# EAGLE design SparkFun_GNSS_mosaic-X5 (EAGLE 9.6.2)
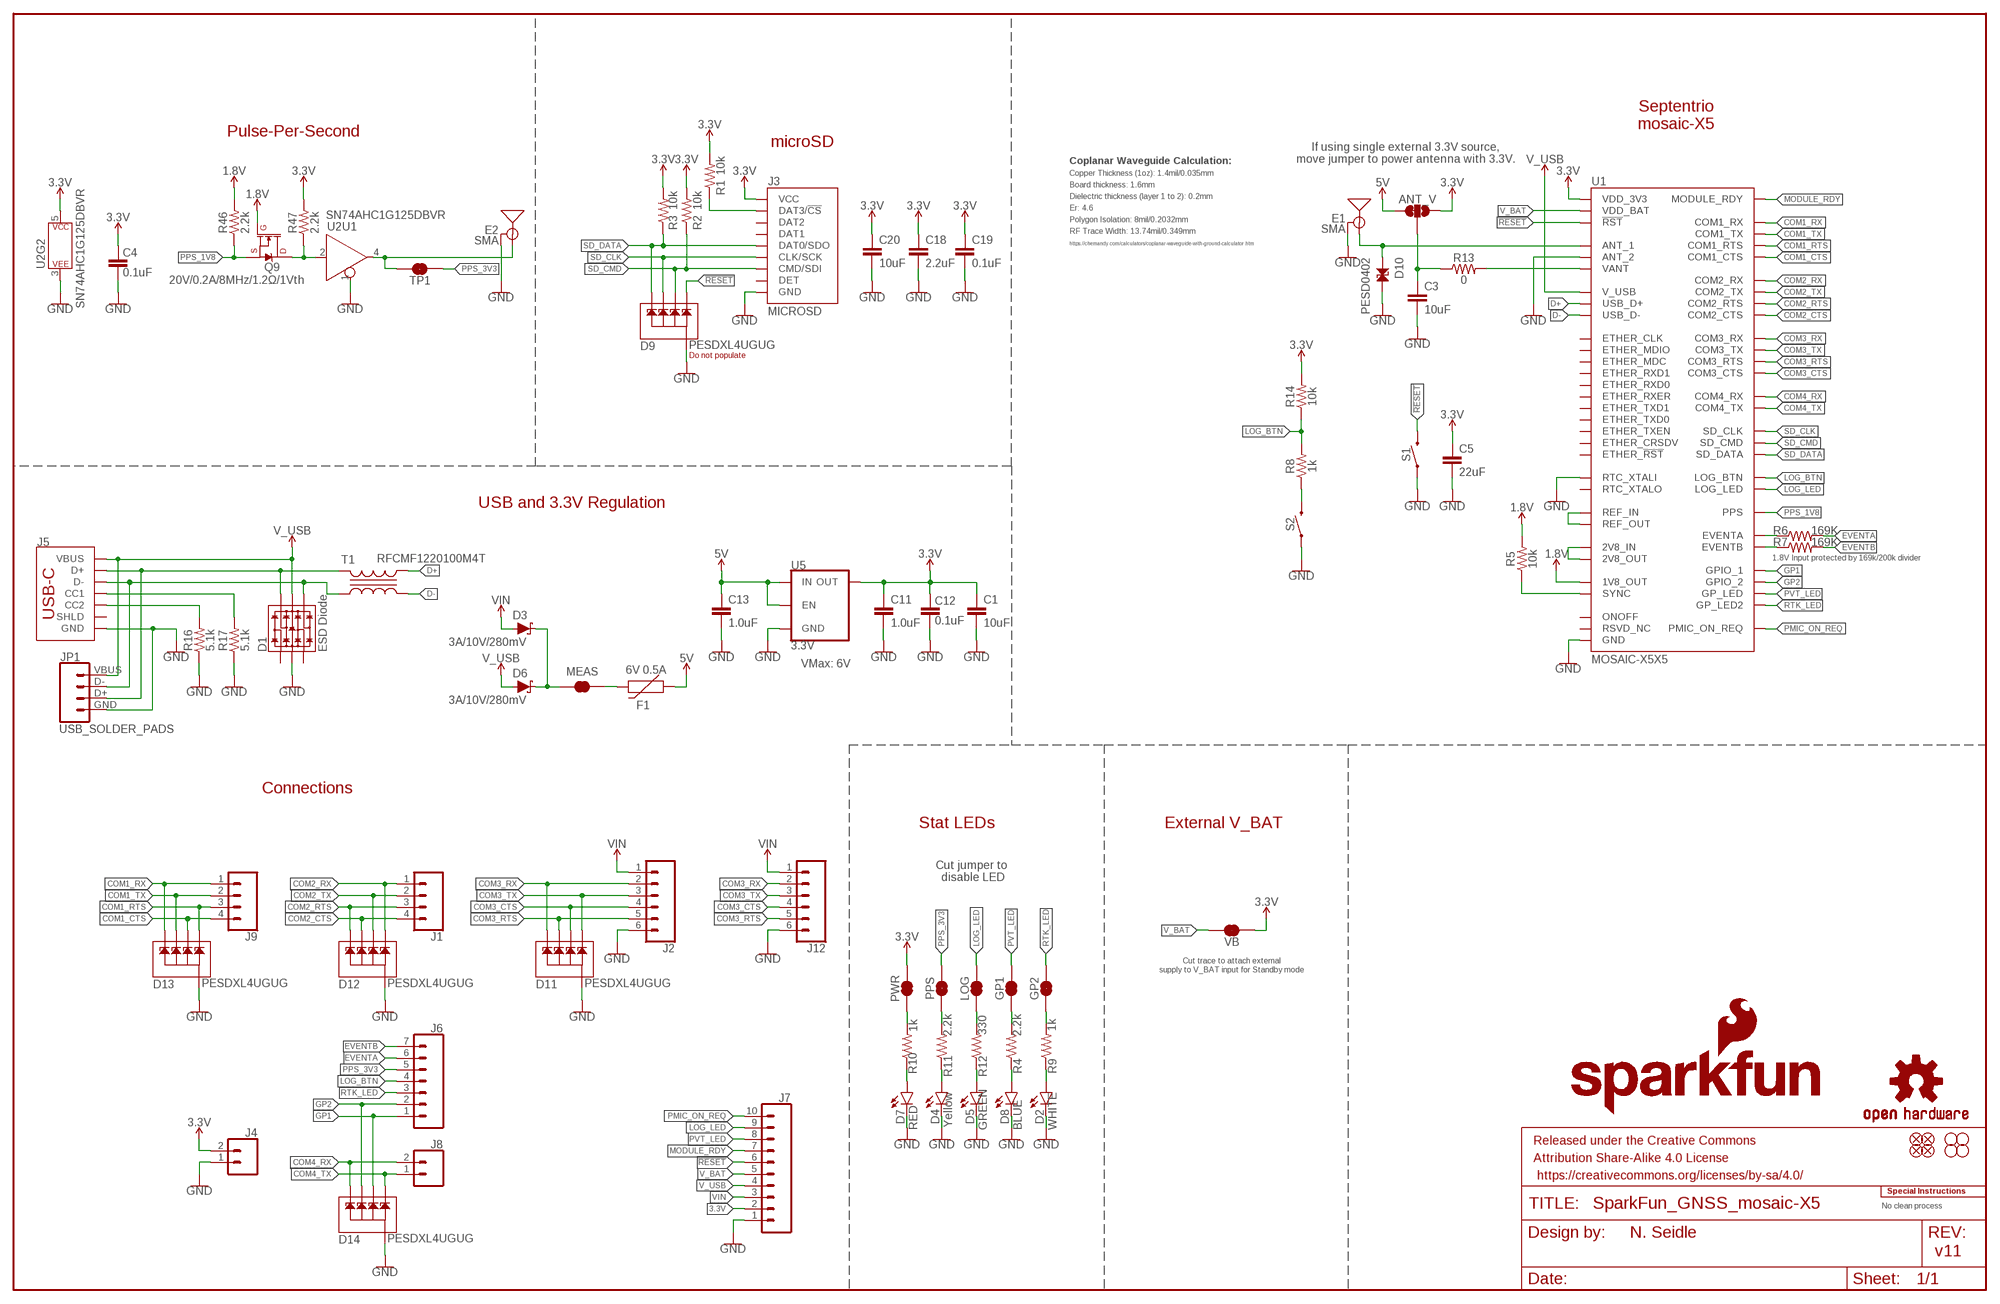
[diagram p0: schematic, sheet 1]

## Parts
ANT_V  JUMPER-SMT_3_1-NC_TRACE_SILK  [SMT-JUMPER_3_1-NC_TRACE_SILK]
C1  10uF  10UF-0603-6.3V-20%  [0603]
C3  10uF  10UF-0603-6.3V-20%  [0603]
C4  0.1uF  0.1UF-0603-25V-5%  [0603]
C5  22uF  22UF-0603-6.3V-20%  [0603]
C11  1.0uF  1.0UF-0603-16V-10%  [0603]
C12  0.1uF  0.1UF-0603-25V-5%  [0603]
C13  1.0uF  1.0UF-0603-16V-10%  [0603]
C18  2.2uF  2.2UF-0603-10V-20%  [0603]
C19  0.1uF  0.1UF-0603-25V-5%  [0603]
C20  10uF  10UF-0603-6.3V-20%  [0603]
D1  ESD Diode  TVS_DIODE_ARRAY_DT1042-04SO-7  [SOT-23-6]
D2  WHITE  LED-WHITE0603  [LED-0603]
D3  3A/10V/280mV  DIODE-SCHOTTKY-BAT60A  [SOD-323]
D4  Yellow  LED-YELLOW0603  [LED-0603]
D5  GREEN  LED-GREEN0603  [LED-0603]
D6  3A/10V/280mV  DIODE-SCHOTTKY-BAT60A  [SOD-323]
D7  RED  LED-RED0603  [LED-0603]
D8  BLUE  LED-BLUE0603  [LED-0603]
D9  PESDXL4UGUG  [SOT353]
D10  PESD0402  PESD0402-0402T  [0402-TIGHT]
D11  PESDXL4UGUG  [SOT353]
D12  PESDXL4UGUG  [SOT353]
D13  PESDXL4UGUG  [SOT353]
D14  PESDXL4UGUG  [SOT353]
E1  SMA  ANTENNA-SMA-GROUNDEDEDGE_SMA  [SMA-EDGE]
E2  SMA  ANTENNA-SMA-GROUNDEDEDGE_SMA  [SMA-EDGE]
F1  6V 0.5A  PPTC_6V500MA  [0805]
FRAME2  FRAME-LEDGER  [CREATIVE_COMMONS]
GP1  JUMPER-SMT_2_NC_TRACE_SILK  [SMT-JUMPER_2_NC_TRACE_SILK]
GP2  JUMPER-SMT_2_NC_TRACE_SILK  [SMT-JUMPER_2_NC_TRACE_SILK]
H1  STAND-OFF  [STAND-OFF]
H2  STAND-OFF  [STAND-OFF]
H3  STAND-OFF  [STAND-OFF]
H4  STAND-OFF  [STAND-OFF]
J1  CONN_041X04_NO_SILK_NO_POP  [1X04_NO_SILK]
J2  CONN_06JST-SMD-LOCKING  [JST-6-SMD-1.25MM-LOCKING]
J3  MICROSD  MICRO-SD-PUSH-PUSH-EXT-PIN  [MICROSD-EXTERNALPIN]
J4  CONN_021X02_NO_SILK  [1X02_NO_SILK]
J5  USB Female Type C Connector  USB_C_4-LAYER_PADS  [USB-C-16P_4LAYER-PADS]
J6  CONN_07NO_SILK  [1X07_NO_SILK]
J7  CONN_10NO_SILK_PTH_FEMALE  [1X10_NO_SILK]
J8  CONN_021X02_NO_SILK  [1X02_NO_SILK]
J9  CONN_041X04_NO_SILK_NO_POP  [1X04_NO_SILK]
J12  CONN_06PAD  [1X06_SOLDER_PADS]
JP1  USB_SOLDER_PADS  [USB-SOLDER-PADS]
JP21  FIDUCIALUFIDUCIAL  [FIDUCIAL-MICRO]
JP61  FIDUCIALUFIDUCIAL  [FIDUCIAL-MICRO]
JP71  FIDUCIALUFIDUCIAL  [FIDUCIAL-MICRO]
JP81  FIDUCIALUFIDUCIAL  [FIDUCIAL-MICRO]
LOG  JUMPER-SMT_2_NC_TRACE_SILK  [SMT-JUMPER_2_NC_TRACE_SILK]
LOGO2  OSHW-LOGOMINI  [OSHW-LOGO-MINI]
LOGO4  SFE_LOGO_NAME_FLAME10_MM  [SFE_LOGO_NAME_FLAME_10MM]
MEAS  JUMPER-COMBO_2_NC_TRACE  [COMBO-JUMPER_2_NC_TRACE]
PPS  JUMPER-SMT_2_NC_TRACE_SILK  [SMT-JUMPER_2_NC_TRACE_SILK]
PWR  JUMPER-SMT_2_NC_TRACE_SILK  [SMT-JUMPER_2_NC_TRACE_SILK]
Q9  20V/0.2A/8MHz/1.2Ω/1Vth  MOSFET-NCH-RE1C002UNTCL  [SOT-416FL]
R1  10k  10KOHM-0603-1/10W-1%  [0603]
R2  10k  10KOHM-0603-1/10W-1%  [0603]
R3  10k  10KOHM-0603-1/10W-1%  [0603]
R4  2.2k  2.2KOHM-0603-1/10W-1%  [0603]
R5  10k  10KOHM-0603-1/10W-1%  [0603]
R6  169K  169KOHM  [0603]
R7  169K  169KOHM  [0603]
R8  1k  1KOHM-0603-1/10W-1%  [0603]
R9  1k  1KOHM-0603-1/10W-1%  [0603]
R10  1k  1KOHM-0603-1/10W-1%  [0603]
R11  2.2k  2.2KOHM-0603-1/10W-1%  [0603]
R12  330  330OHM-0603-1/10W-1%  [0603]
R13  0  0OHM-0603-1/10W  [0603]
R14  10k  10KOHM-0603-1/10W-1%  [0603]
R16  5.1k  5.1KOHM5.1KOHM-0603-1/10W-1%  [0603]
R17  5.1k  5.1KOHM5.1KOHM-0603-1/10W-1%  [0603]
R46  2.2k  2.2KOHM-0603-1/10W-1%  [0603]
R47  2.2k  2.2KOHM-0603-1/10W-1%  [0603]
S1  MOMENTARY-SWITCH-SPST-SMD-4.6X2.8MM  [TACTILE_SWITCH_SMD_4.6X2.8MM]
S2  MOMENTARY-SWITCH-SPST-SMD-5.2-TALL-REDUNDANT  [TACTILE_SWITCH_SMD_5.2MM]
T1  RFCMF1220100M4T  TRANSFORMER0508  [RFCMF1220100M4T]
TP1  JUMPER-SMT_2_NC_TRACE_SILK  [SMT-JUMPER_2_NC_TRACE_SILK]
U1  MOSAIC-X5X5  [MOSAIC_LGA]
U2  SN74AHC1G125DBVR  74AHC1G125SN74AHC1G125DBVR  [SOT23-5]
U5  3.3V  V_REG_AP2112K-3.3V  [SOT23-5]
U$2  SPECIAL_INSTRUCTIONS-ORDERING  [ORDERING_INSTRUCTIONS]
VB  JUMPER-SMT_2_NC_TRACE_SILK  [SMT-JUMPER_2_NC_TRACE_SILK]

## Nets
1.8V: Q9.1(G) R5.2 R46.2 U1.AC4(1V8_OUT)
3.3V [power]: ANT_V.1 C1.1 C4.2 C5.1 C11.1 C12.2 C18.1 C19.1 C20.1 J3.4(VCC) J4.2 J7.2 PWR.2 R1.2 R2.2 R3.2 R14.2 R47.2 U1.A18(VDD_3V3) U1.A19(VDD_3V3) U1.A20(VDD_3V3) U1.B18(VDD_3V3) U1.B19(VDD_3V3) U1.B20(VDD_3V3) U1.C18(VDD_3V3) U1.C19(VDD_3V3) U1.C20(VDD_3V3) U2.5(P$V+) U5.5(OUT) VB.1
5V: ANT_V.3 C13.1 F1.1 U5.1(IN) U5.3(EN)
!RESET!: D9.3 J7.6 S1.3 S1.4 U1.A11(!RST!)
ANT_V: ANT_V.2 C3.1 R13.1
CC1: J5.A5(CC1) R17.2
CC2: J5.B5(CC2) R16.2
COM1_CTS: D13.4 J9.4 U1.E1(COM1_CTS)
COM1_RTS: D13.3 J9.3 U1.C1(COM1_RTS)
COM1_RX: D13.1 J9.1 U1.B1(COM1_RX)
COM1_TX: D13.5 J9.2 U1.D1(COM1_TX)
COM2_CTS: D12.5 J1.4 U1.J1(COM2_CTS)
COM2_RTS: D12.1 J1.3 U1.G1(COM2_RTS)
COM2_RX: D12.3 J1.1 U1.F1(COM2_RX)
COM2_TX: D12.4 J1.2 U1.H1(COM2_TX)
COM3_CTS: D11.4 J2.4 J12.4 U1.N1(COM3_CTS)
COM3_RTS: D11.5 J2.5 J12.5 U1.L1(COM3_RTS)
COM3_RX: D11.1 J2.2 J12.2 U1.K1(COM3_RX)
COM3_TX: D11.3 J2.3 J12.3 U1.M1(COM3_TX)
COM4_RX: D14.1 J8.2 U1.D3(COM4_RX)
COM4_TX: D14.3 J8.1 U1.E3(COM4_TX)
D+: T1.B2 U1.A5(USB_D+)
D-: T1.A2 U1.A6(USB_D-)
EVENTA: J6.6 R6.2
EVENTB: J6.7 R7.2
GND: C1.2 C3.2 C4.1 C5.2 C11.2 C12.1 C13.2 C18.2 C19.2 C20.2 D1.2(VSS) D2.C D4.C D5.C D7.C D8.C D9.2 D10.2 D11.2 D12.2 D13.2 D14.2 E1.GND@0(GND) E1.GND@1(GND) E1.GND@2(GND) E1.GND@3(GND) E2.GND@0(GND) E2.GND@1(GND) E2.GND@2(GND) E2.GND@3(GND) J2.6 J3.6(GND) J3.10(GND) J3.11(GND) J3.12(GND) J3.13(GND) J4.1 J5.GND J5.GND2(GND) J7.1 J12.6 JP1.GND R16.1 R17.1 S1.1 S1.2 S2.1 S2.2 U1.A3(RTC_XTALI) U1.A4(GND) U1.A7(GND) U1.A15(GND) U1.A16(GND) U1.A17(GND) U1.A21(GND) U1.A22(GND) U1.A23(GND) U1.AA13(GND) U1.AA14(GND) U1.AA15(GND) U1.AA16(GND) U1.AA17(GND) U1.AA18(GND) U1.AA19(GND) U1.AA20(GND) U1.AA21(GND) U1.AA22(GND) U1.AA23(GND) U1.AB2(GND) U1.AB3(GND) U1.AB4(GND) U1.AB5(GND) U1.AB6(GND) U1.AB7(GND) U1.AB8(GND) U1.AB13(GND) U1.AB14(GND) U1.AB15(GND) U1.AB16(GND) U1.AB17(GND) U1.AB18(GND) U1.AB19(GND) U1.AB20(GND) U1.AB21(GND) U1.AB22(GND) U1.AB23(GND) U1.AC13(GND) U1.AC15(GND) U1.AC18(GND) U1.AC19(GND) U1.AC21(GND) U1.AC22(GND) U1.AC23(GND) U1.B4(GND) U1.B5(GND) U1.B6(GND) U1.B7(GND) U1.B13(GND) U1.B17(GND) U1.B21(GND) U1.C4(GND) U1.C7(GND) U1.C15(GND) U1.C16(GND) U1.C17(GND) U1.C23(GND) U1.D2(GND) U1.D21(GND) U1.D22(GND) U1.D23(GND) U1.E2(GND) U1.E21(GND) U1.E22(GND) U1.E23(GND) U1.F21(GND) U1.F22(GND) U1.F23(GND) U1.G2(GND) U1.G21(GND) U1.G23(GND) U1.H21(GND) U1.H22(GND) U1.H23(GND) U1.J21(GND) U1.J22(GND) U1.J23(GND) U1.K2(GND) U1.K21(GND) U1.K22(GND) U1.K23(GND) U1.L21(GND) U1.L22(GND) U1.L23(GND) U1.M21(GND) U1.M22(GND) U1.N21(GND) U1.N22(GND) U1.P1(GND) U1.P2(GND) U1.P3(GND) U1.P21(GND) U1.P22(GND) U1.R3(GND) U1.R21(GND) U1.R22(GND) U1.T21(GND) U1.T22(GND) U1.T23(GND) U1.U2(GND) U1.U21(GND) U1.U22(GND) U1.U23(GND) U1.V21(GND) U1.V22(GND) U1.V23(ANT_2) U1.W21(GND) U1.W22(GND) U1.W23(GND) U1.Y2(GND) U1.Y21(GND) U1.Y22(GND) U1.Y23(GND) U2.1(U1:!EN) U2.3(P$V-) U5.2(GND)
GP1: D14.4 J6.1 U1.AA4(GPIO_1)
GP2: D14.5 J6.2 U1.L3(GPIO_2)
GPS_ANT1 [RF]: D10.1 E1.SIG(SIGNAL) U1.AC20(ANT_1)
LOG_BTN: J6.4 R8.2 R14.1 U1.K3(LOG_BTN)
LOG_LED: J7.9 LOG.2 U1.B2(LOG_LED)
MEAS: D3.C D6.C MEAS.2 MEAS.4
MODULE_RDY: J7.7 U1.A12(MODULE_RDY)
N$1: R8.1 S2.3 S2.4
N$2: D4.A R11.1
N$3: PPS.1 R11.2
N$4: F1.2 MEAS.1 MEAS.3
N$5: J3.2(DAT3/!CS!) R1.1
N$6: R6.1 U1.AC6(EVENTA)
N$7: R7.1 U1.AC7(EVENTB)
N$8: D2.A R9.1
N$9: GP2.1 R9.2
N$10: U1.AC16(REF_OUT) U1.AC17(REF_IN)
N$11: D8.A R4.1
N$12: GP1.1 R4.2
N$14: D7.A R10.1
N$15: U1.M23(2V8_IN) U1.N23(2V8_OUT)
N$16: D5.A R12.1
N$17: LOG.1 R12.2
N$20: PWR.1 R10.2
N$26: R5.1 U1.AC3(SYNC)
PMIC_ON_REQ: J7.10 U1.B16(PMIC_ON_REQ)
PPS: E2.SIG(SIGNAL) TP1.2 U2.4(U1:Y)
PPS_1V8: Q9.2(S) R46.1 U1.AC8(PPS)
PPS_3: Q9.3(D) R47.1 U2.2(U1:A)
PPS_3V3: J6.5 PPS.2 TP1.1
PVT_LED: GP1.2 J7.8 U1.A14(GP_LED)
RTK_LED: GP2.2 J6.3 U1.M3(GP_LED2)
SD_CLK: D9.5 J3.5(CLK/SCK) U1.AA1(SD_CLK)
SD_CMD: D9.4 J3.3(CMD/SDI) R2.1 U1.AB1(SD_CMD)
SD_DATA: D9.1 J3.7(DAT0/SDO) R3.1 U1.Y1(SD_DATA)
USB_D+: D1.6(IO4) J5.A6(D+) J5.B6(D+) JP1.D+ T1.B1
USB_D-: D1.4(IO3) J5.A7(D-) J5.B7(D-) JP1.D- T1.A1
V_BAT: J7.5 U1.B8(VDD_BAT) VB.2
V_USB: D1.5(VCC) D6.A J5.VBUS1(VBUS) J5.VBUS2(VBUS) J7.4 JP1.VBUS U1.A8(V_USB)
VANT: R13.2 U1.P23(VANT) U1.R23(VANT)
VIN: D3.A J2.1 J7.3 J12.1
Unconnected: D1.1(IO1) D1.3(IO2) J3.1(DAT2) J3.8(DAT1) J3.9(DET) J5.SHLD1(SHLD) J5.SHLD2(SHLD) J5.SHLD3(SHLD) J5.SHLD4(SHLD) U1.A2(RTC_XTALO) U1.A9(RSVD_NC) U1.A10(ONOFF) U1.A13(RSVD_NC) U1.AA2(ETHER_CLK) U1.AA3(RSVD_NC) U1.AA5(RSVD_NC) U1.AA6(RSVD_NC) U1.AA7(RSVD_NC) U1.AA8(RSVD_NC) U1.AA9(RSVD_NC) U1.AA10(RSVD_NC) U1.AA11(RSVD_NC) U1.AA12(RSVD_NC) U1.AB9(RSVD_NC) U1.AB10(RSVD_NC) U1.AB11(RSVD_NC) U1.AB12(RSVD_NC) U1.AC1(RSVD_NC) U1.AC2(RSVD_NC) U1.AC5(RSVD_NC) U1.AC9(RSVD_NC) U1.AC10(RSVD_NC) U1.AC11(RSVD_NC) U1.AC12(RSVD_NC) U1.AC14(RSVD_NC) U1.B3(RSVD_NC) U1.B9(RSVD_NC) U1.B10(RSVD_NC) U1.B11(RSVD_NC) U1.B12(RSVD_NC) U1.B14(RSVD_NC) U1.B15(RSVD_NC) U1.B22(RSVD_NC) U1.B23(RSVD_NC) U1.C2(RSVD_NC) U1.C3(RSVD_NC) U1.C5(RSVD_NC) U1.C6(RSVD_NC) U1.C8(RSVD_NC) U1.C9(RSVD_NC) U1.C10(RSVD_NC) U1.C11(RSVD_NC) U1.C12(RSVD_NC) U1.C13(RSVD_NC) U1.C14(RSVD_NC) U1.C21(RSVD_NC) U1.C22(RSVD_NC) U1.F2(ETHER_!RST!) U1.F3(RSVD_NC) U1.G3(RSVD_NC) U1.G22(RSVD_NC) U1.H2(ETHER_TXD1) U1.H3(RSVD_NC) U1.J2(ETHER_TXD0) U1.J3(RSVD_NC) U1.L2(ETHER_TXEN) U1.M2(ETHER_RXER) U1.N2(ETHER_CRSDV) U1.N3(RSVD_NC) U1.R1(RSVD_NC) U1.R2(ETHER_RXD0) U1.T1(RSVD_NC) U1.T2(ETHER_RXD1) U1.T3(RSVD_NC) U1.U1(RSVD_NC) U1.U3(RSVD_NC) U1.V1(RSVD_NC) U1.V2(ETHER_MDC) U1.V3(RSVD_NC) U1.W1(RSVD_NC) U1.W2(ETHER_MDIO) U1.W3(RSVD_NC) U1.Y3(RSVD_NC)

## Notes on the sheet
- Septentrio
  mosaic-X5
- Pulse-Per-Second
- microSD
- If using single external 3.3V source,
  move jumper to power antenna with 3.3V.
- Coplanar Waveguide Calculation:
- Copper Thickness (1oz): 1.4mil/0.035mm
- Board thickness: 1.6mm
- Dielectric thickness (layer 1 to 2): 0.2mm
- Er: 4.6
- Polygon Isolation: 8mil/0.2032mm
- RF Trace Width: 13.74mil/0.349mm
- https://chemandy.com/calculators/coplanar-waveguide-with-ground-calculator.htm
- Do not populate
- USB and 3.3V Regulation
- 1.8V Input protected by 169k/200k divider
- VMax: 6V
- Connections
- Stat LEDs | External V_BAT
- Cut jumper to 
  disable LED
- Cut trace to attach external
  supply to V_BAT input for Standby mode
- No clean process
- N. Seidle
- v11

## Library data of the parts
ANT_V = SparkFun-Jumpers:JUMPER-SMT_3_1-NC_TRACE: Normally closed trace jumper (1 of 2 connections) This jumper has a trace between two pads so it's normally closed (NC). The other connection is normally open (NO). Use a razor knife to open the connection. For best results follow the IPC guidelines for cutting traces: Cutout at least 0.063 mm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
C1 C3 C20 = SparkFun-Capacitors:10UF: 10.0µF ceramic capacitors; PROD_ID: CAP-11015
C4 C12 C19 = SparkFun-Capacitors:0.1UF: 0.1µF ceramic capacitors; PROD_ID: CAP-08604
C5 = SparkFun-Capacitors:22UF: 22µF ceramic capacitors; PROD_ID: CAP-14464
C11 C13 = SparkFun-Capacitors:1.0UF: 1µF ceramic capacitors; PROD_ID: CAP-00868
C18 = SparkFun-Capacitors:2.2UF: 2.2µF ceramic capacitors; PROD_ID: CAP-07888
D1 = SparkFun-DiscreteSemi:TVS_DIODE_ARRAY; PROD_ID: IC-13538
D2 = SparkFun-LED:LED-WHITE: White SMD LED; PROD_ID: DIO-09004
D3 D6 = SparkFun-DiscreteSemi:DIODE-SCHOTTKY: Schottky diode; PROD_ID: DIO-14072
D4 = SparkFun-LED:LED-YELLOW: Yellow SMD LED; PROD_ID: DIO-09003
D5 = SparkFun-LED:LED-GREEN: Green SMD LED; PROD_ID: DIO-00821
D7 = SparkFun-LED:LED-RED: Red SMD LED; PROD_ID: DIO-00819
D8 = SparkFun-LED:LED-BLUE: Blue SMD LED; PROD_ID: DIO-08575
D9 D11-D14 = SparkFun-DiscreteSemi:PESDXL4UG; PROD_ID: DIO-19494
D10 = SparkFun-DiscreteSemi:PESD0402: ESD protection diode; PROD_ID: DIO-15359
E1 E2 = SparkFun-RF:ANTENNA-SMA-GROUNDED: SMA Antenna Connector w/ Ground; PROD_ID: CONN-08289
F1 = SparkFun-Fuses:PPTC: Resettable Fuse PPTC; PROD_ID: RES-13945
FRAME2 = SparkFun-Aesthetics:FRAME-LEDGER: Schematic Frame - Ledger
GP1 GP2 LOG PPS PWR TP1 VB = SparkFun-Jumpers:JUMPER-SMT_2_NC_TRACE: Normally closed trace jumper
H1-H4 = SparkFun-Hardware:STAND-OFF: Stand Off
J1 J9 = SparkFun-Connectors:CONN_04: Multi connection point. Often used as Generic Header-pin footprint for 0.1 inch spaced/style header connections On any of the 0.1 inch spaced packages, you can populate with these: Break Away Headers - Straight (PRT-00116) Break Away Male Headers - Right Angle (PRT-00553) Female Headers (PRT-00115)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
J2 = SparkFun-Connectors:CONN_06: Multi connection point. Often used as Generic Header-pin footprint for 0.1 inch spaced/style header connections On any of the 0.1 inch spaced packages, you can populate with these: Break Away Headers - Straight (PRT-00116) Break Away Male Headers - Right Angle (PRT-00553) Female Headers (PRT-00115)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; PROD_ID: CONN-16497
J3 = SparkFun-Connectors:MICRO-SD: microSD Socket for Transflash Various sockets for µSD. tDoc lines correctly indicate media card edge positions when inserting (unlocked, locked, depressed). NOTE: CD1 and CD2 are connected internally, and the default detect state of the socket is detect pin to ground. SparkFun Products: WAV Trigger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; PROD_ID: CONN-16110
J4 J8 = SparkFun-Connectors:CONN_02: Multi connection point. Often used as Generic Header-pin footprint for 0.1 inch spaced/style header connections
J5 = SparkFun-Connectors:USB_C: USB Type C 16Pin Connector Super Speed pins not available on the 16-pin purely SMD connector so this part is best for USB 2.0 implementations. D1 and D2 are tied together enabling D+/- no matter which way the cable is plugged into the connector. The two channel configuration pins (CC1/2) are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; PROD_ID: CONN-14122
J6 = SparkFun-Connectors:CONN_07: Multi connection point. Often used as Generic Header-pin footprint for 0.1 inch spaced/style header connections On any of the 0.1 inch spaced packages, you can populate with these: Break Away Headers - Straight (PRT-00116) Break Away Male Headers - Right Angle (PRT-00553) Female Headers (PRT-00115)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
J7 = SparkFun-Connectors:CONN_10: Multi connection point. Often used as Generic Header-pin footprint for 0.1 inch spaced/style header connections On any of the 0.1 inch spaced packages, you can populate with these: Break Away Headers - Straight (PRT-00116) Break Away Male Headers - Right Angle (PRT-00553) Female Headers (PRT-00115)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
J12 = SparkFun-Connectors:CONN_06: Multi connection point. Often used as Generic Header-pin footprint for 0.1 inch spaced/style header connections On any of the 0.1 inch spaced packages, you can populate with these: Break Away Headers - Straight (PRT-00116) Break Away Male Headers - Right Angle (PRT-00553) Female Headers (PRT-00115)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
JP1 = SparkFun-Connectors:USB_SOLDER_PADS: Solder pad access to USB pins. Helpful to expose on PCBs so user can attach external USB connector if necessary.
JP21 JP61 JP71 JP81 = SparkFun-Aesthetics:FIDUCIAL: Fiducial Alignment Points
LOGO2 = SparkFun-Aesthetics:OSHW-LOGO: Open-Source Hardware (OSHW) Logo
LOGO4 = SparkFun-Aesthetics:SFE_LOGO_NAME_FLAME: SparkFun Font Logo w/ Flame
MEAS = SparkFun-Jumpers:JUMPER-COMBO_2_NC_TRACE
Q9 = SparkFun-DiscreteSemi:MOSFET-NCH: N-channel MOSFETs Voltage controlled devices that allow control of high current outputs. SparkFun Products: SparkFun OpenScale SparkFun Digital Sandbox SparkFun Monster Moto Shield SparkFun MOSFET Power Controller; PROD_ID: TRANS-14399
R1-R3 R5 R14 = SparkFun-Resistors:10KOHM: 10kΩ resistor; PROD_ID: RES-00824
R4 R11 R46 R47 = SparkFun-Resistors:2.2KOHM: 2.2kΩ resistor; PROD_ID: RES-08272
R6 R7 = SparkFun-Resistors:169KOHM: 169kΩ resistor; PROD_ID: RES-14394
R8-R10 = SparkFun-Resistors:1KOHM: 1kΩ resistor; PROD_ID: RES-07856
R12 = SparkFun-Resistors:330OHM: 330Ω resistor; PROD_ID: RES-00818
R13 = SparkFun-Resistors:0OHM: 0Ω resistor; PROD_ID: RES-08609
R16 R17 = SparkFun-Resistors:5.1KOHM; PROD_ID: RES-12083
S1 = SparkFun-Switches:MOMENTARY-SWITCH-SPST: Momentary Switch (Pushbutton) - SPST; PROD_ID: SWCH-15606
S2 = SparkFun-Switches:MOMENTARY-SWITCH-SPST: Momentary Switch (Pushbutton) - SPST; PROD_ID: SWCH-14139
T1 = SparkFun-Coils:TRANSFORMER: Small transformers; PROD_ID: COMP-19495
U1 = Septentrio_mosaic-X5:MOSAIC-X5; PROD_ID: GPS-19395
U2 = SparkFun-IC-Logic:74*1G125: Single buffer Buffers & Line Drivers Tri-State Single Bus SOT-23-5 Datasheet SparkFun Products SparkFun SAMD21 Mini Breakout (DEV-13664) SparkFun SAMD21 Dev Breakout (DEV-13672) SparkFun MIDI Shield (DEV-12898) SparkFun WiFi Shield - CC3000 (DEV-12071) SparkFun Tsunami Super WAV Trigger (Qwiic)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; PROD_ID: IC-11920
U5 = SparkFun-IC-Power:V_REG_AP2112: AP2112 - 600mA CMOS LDO Regulator w/ Enable The AP2112 is CMOS process low dropout linear regulator with enable function, the regulator delivers a guaranteed 600mA (min.) continuous load current. Features Output Voltage Accuracy: ±1.5% Output Current: 600mA (Min.) Foldback Short Current Protection: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; PROD_ID: VREG-12457
U$2 = SparkFun-Aesthetics:SPECIAL_INSTRUCTIONS: Special Ordering/Production Instructions Alert

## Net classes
1 power: width 0.178 mm
2 3.3V: width 0.508 mm, drill 0.305 mm
3 RF: width 0.349 mm, clearance 0.203 mm

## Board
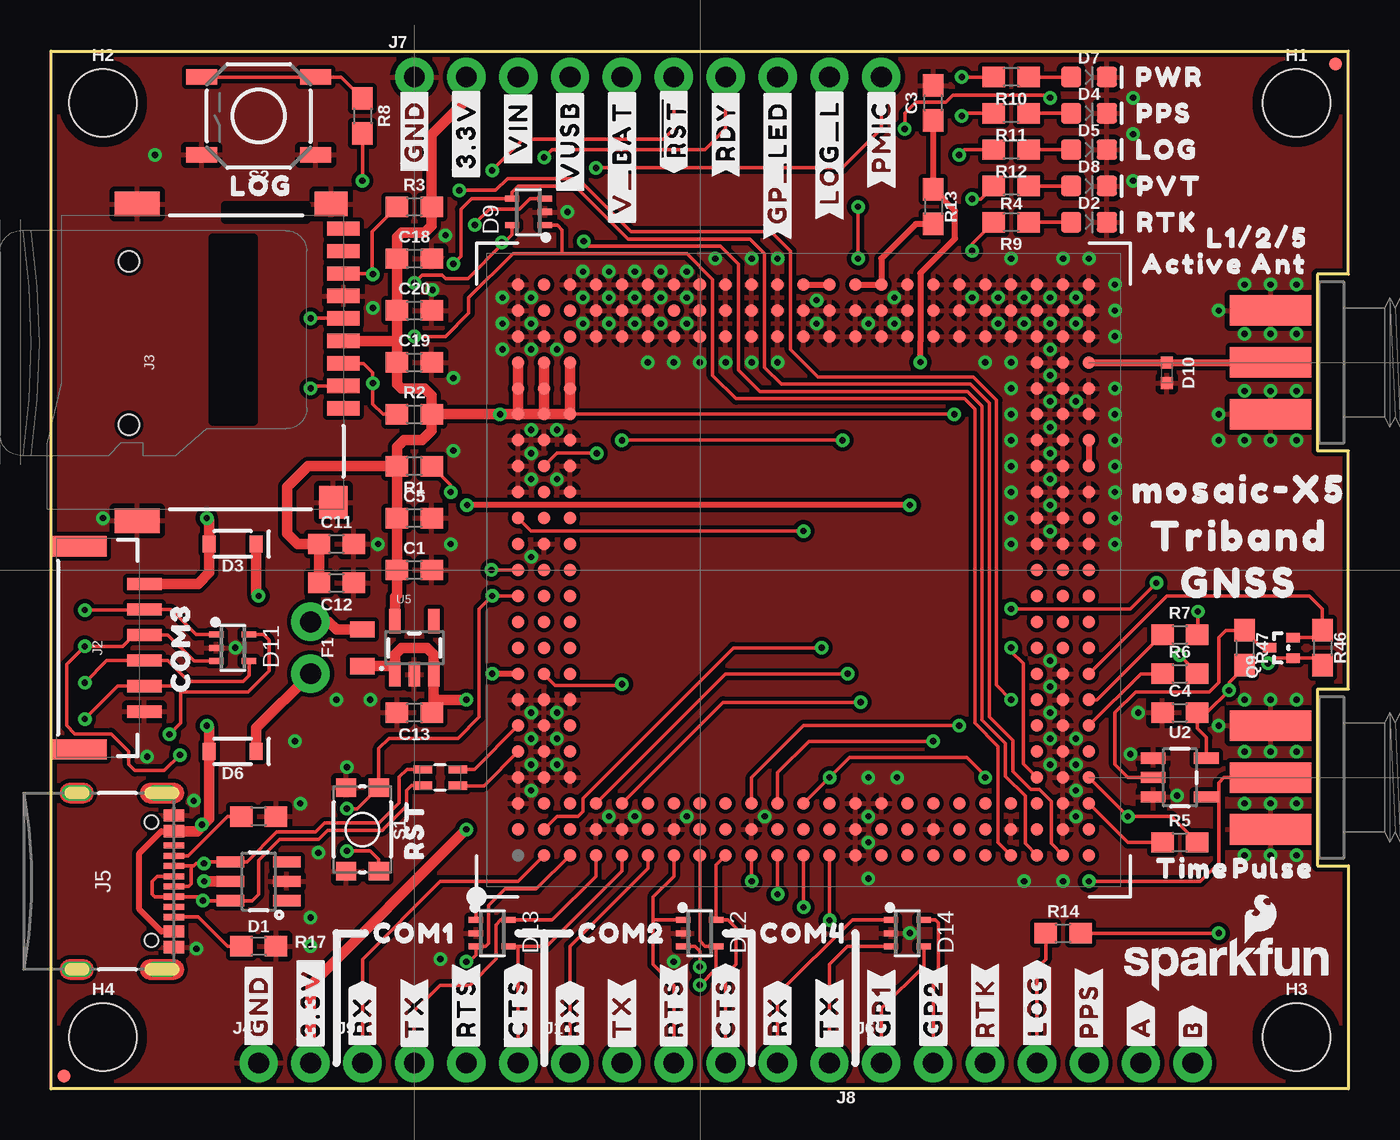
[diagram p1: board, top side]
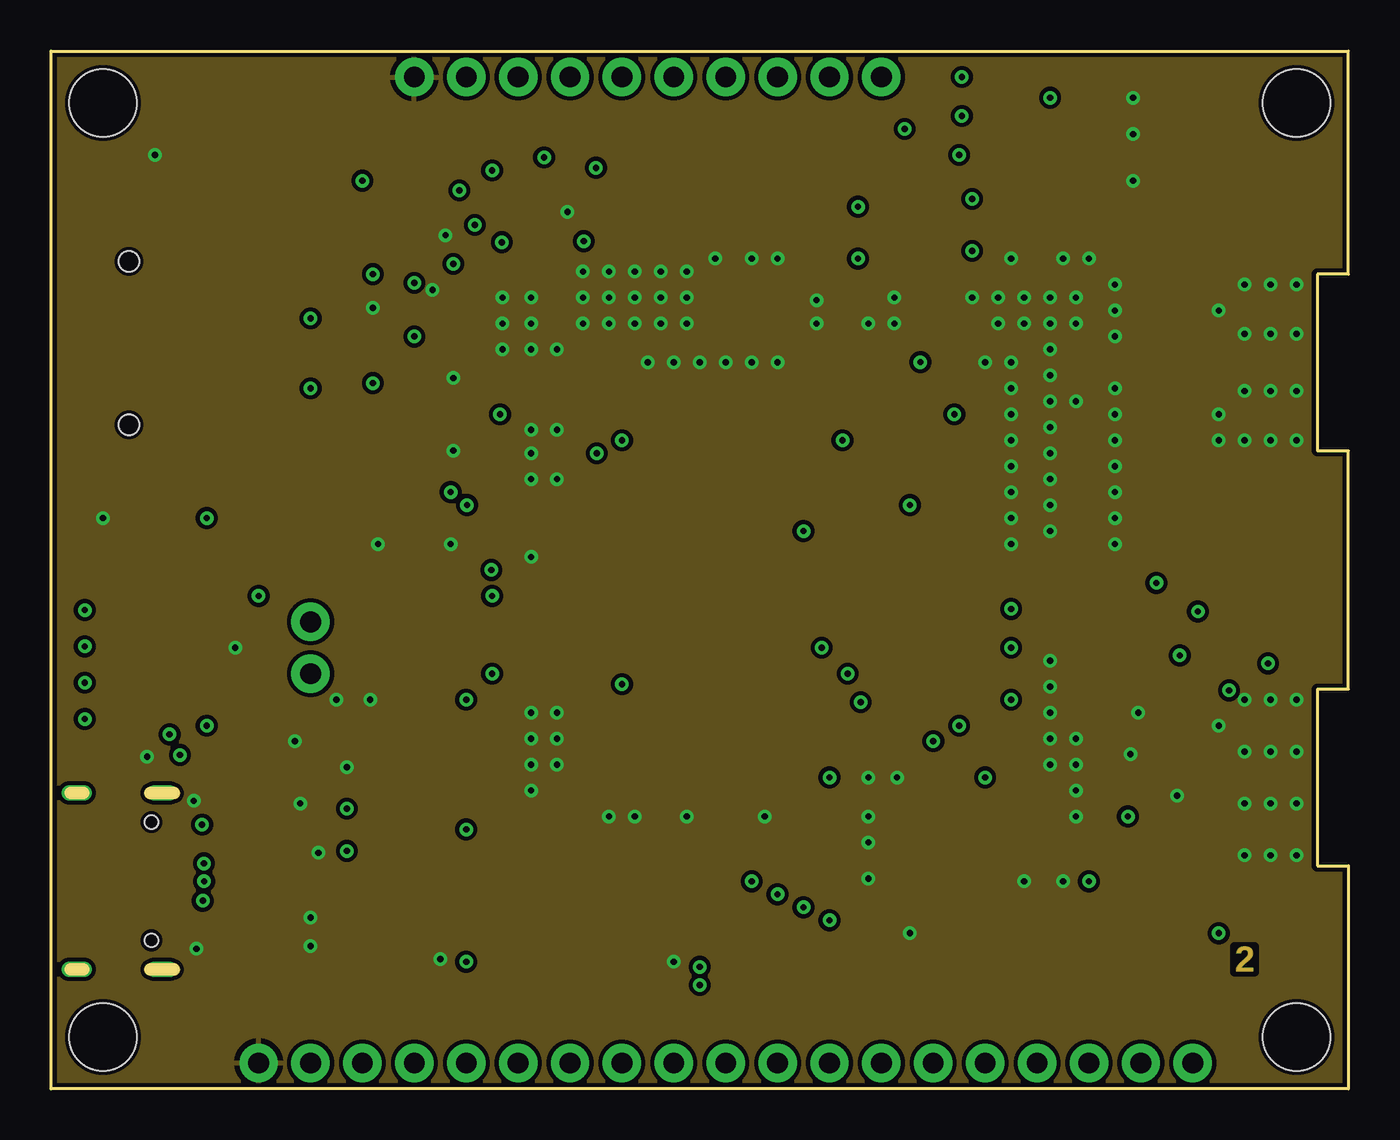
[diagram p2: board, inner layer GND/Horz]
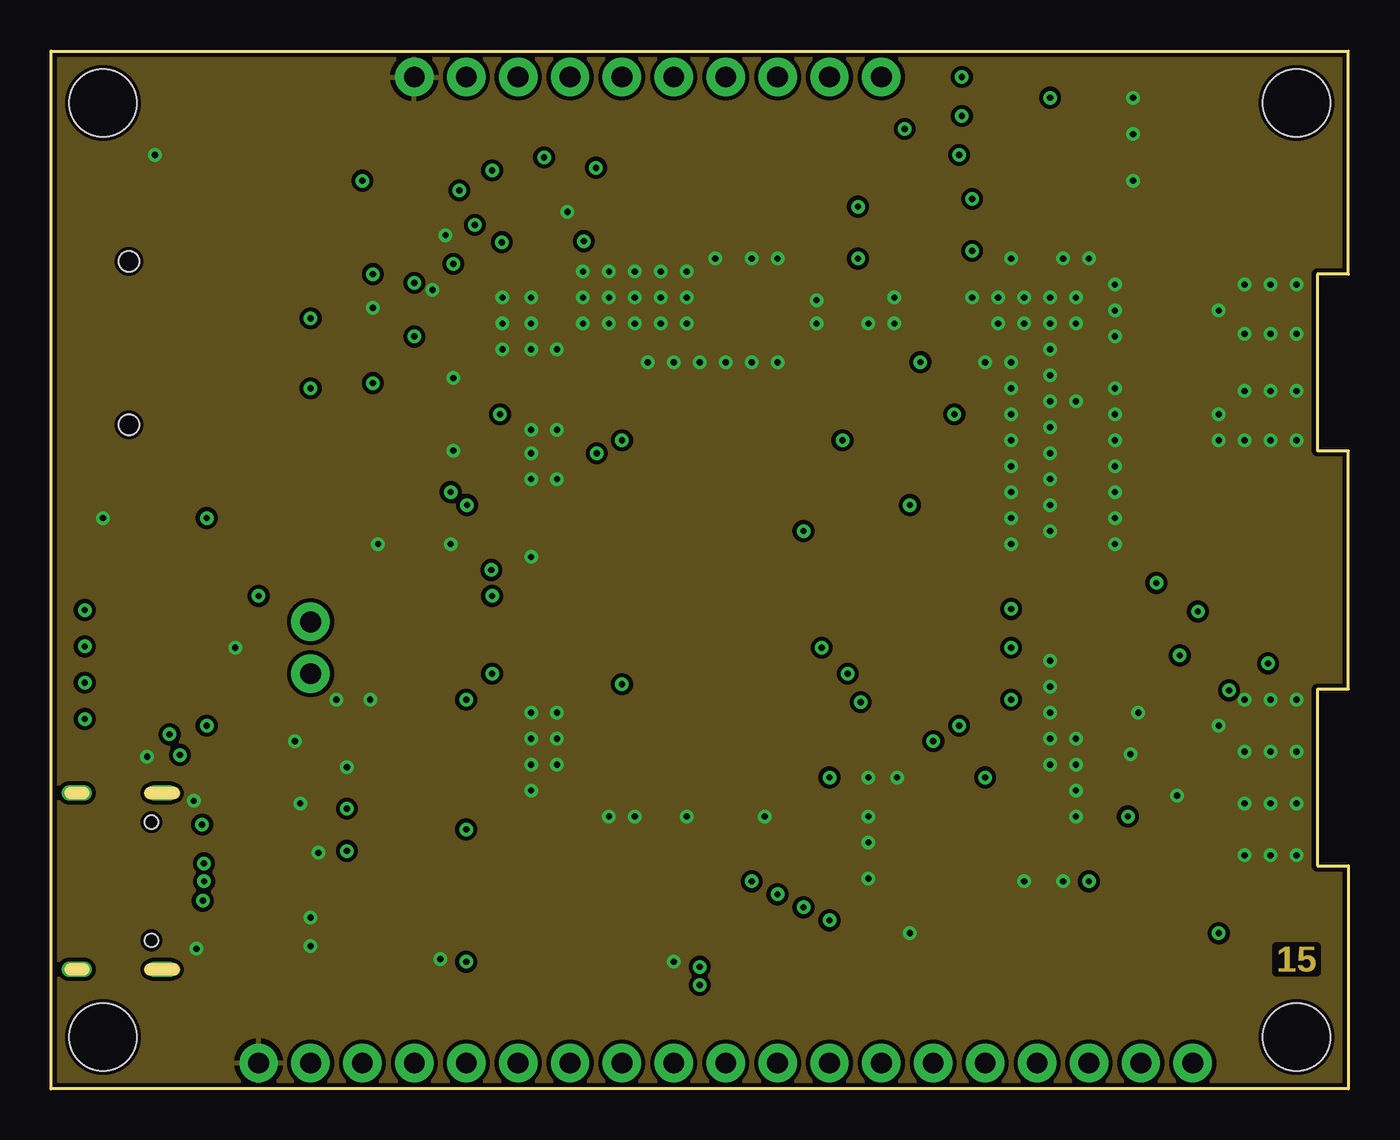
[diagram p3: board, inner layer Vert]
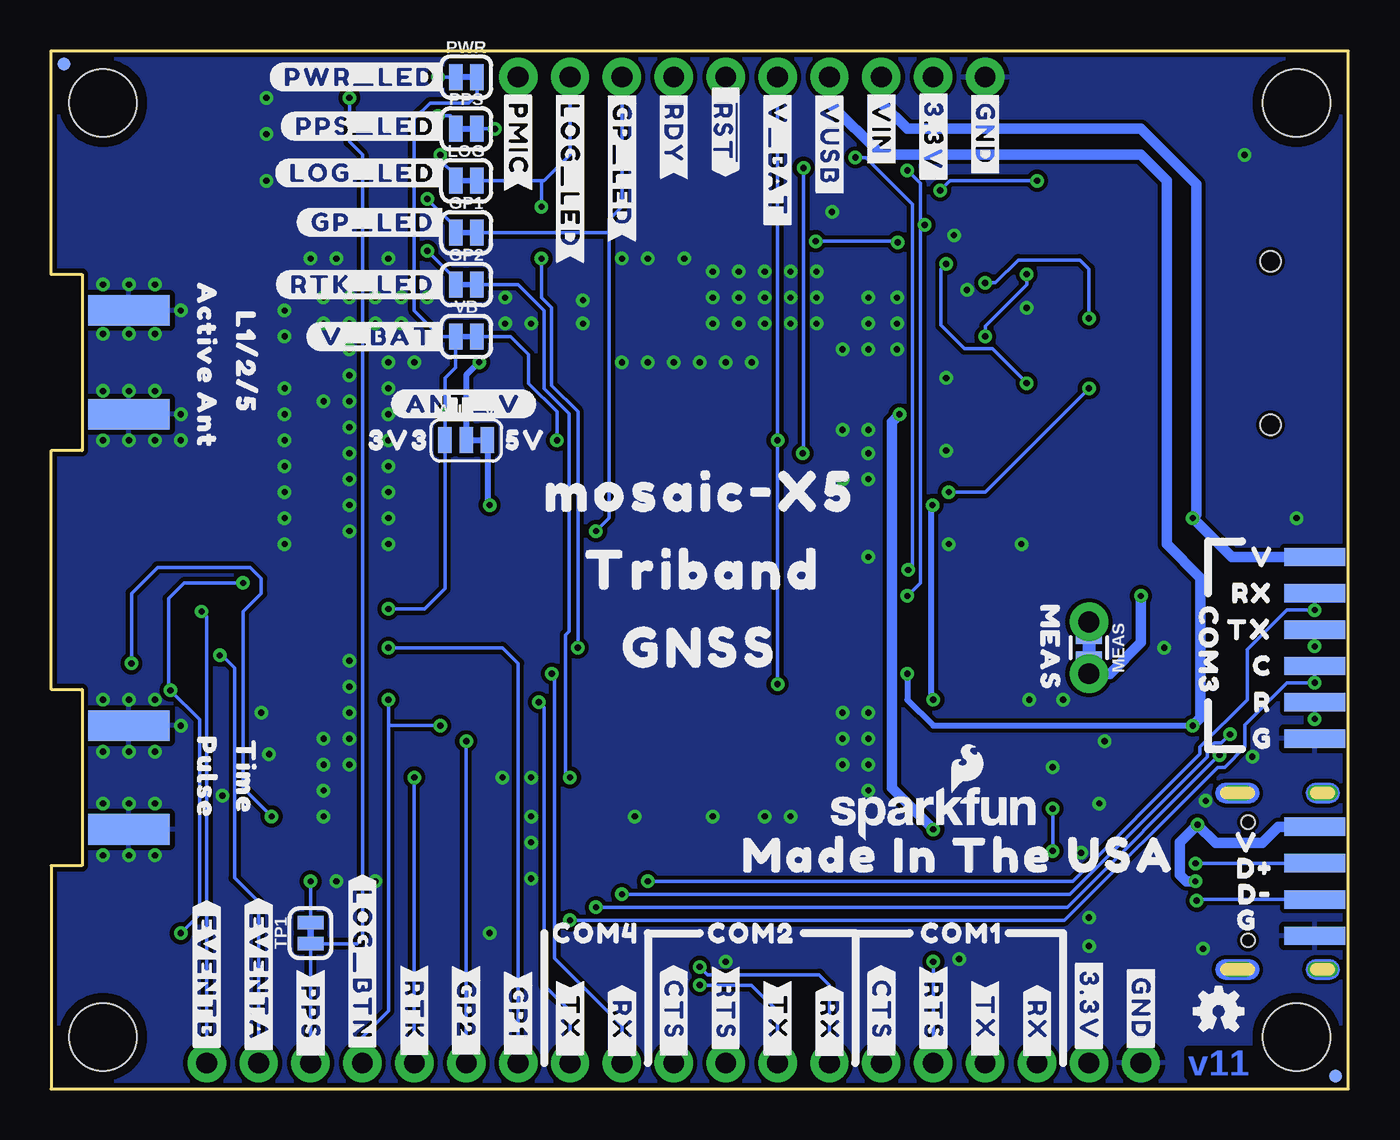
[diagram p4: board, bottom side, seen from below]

Size 63.5 x 50.8 mm. Coordinates in mm from the lower left corner, seen from the top.
Outline: 0,0 0,50.8 63.5,50.8 63.5,39.88 61.98,39.88 61.98,31.24 63.5,31.24 63.5,19.56 61.98,19.56 61.98,10.92 63.5,10.92 63.5,0 0,0
Copper layers (1+2*15+16): Top/Horz 0.035559375mm / dielectric 0.47751875mm / GND/Horz 0.035559375mm / dielectric 0.47751875mm / Vert 0.035559375mm / dielectric 0.47751875mm / Bottom/Vert 0.035559375mm
Design rules "SparkFun-4-Layer-General-JLCPCB": minimum track width 7mil, minimum drill 12mil, track to track 7mil, track to pad 7mil, pad to pad 7mil, via to via 7mil, smd to smd 7mil, copper to edge 7mil, drill to drill 7mil, minimum pad ring 7mil, minimum via ring 7mil, stop-mask expansion 3mil, vias tented up to drill 25mil, thermal gap 10mil

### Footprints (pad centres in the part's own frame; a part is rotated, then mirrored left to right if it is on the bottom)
SMT-JUMPER_3_1-NC_TRACE_SILK = smd 0.66 x 1.27: 1 -1.041,0; 2 0,0; 3 1.041,0
0603 = smd 1.1 x 1: 1 -0.85,0; 2 0.85,0
SOT-23-6 = smd 0.55 x 1.35: 1 -0.95,-1.375; 2 0,-1.375; 3 0.95,-1.375; 4 0.95,1.375; 5 0,1.375; 6 -0.95,1.375
LED-0603 = smd 1 x 1: A -0.877,0; C 0.877,0
SOD-323 = smd 0.63 x 0.83: A 1.15,0; C -1.15,0
SOT353 = smd 0.3 x 0.7: 1 -0.65,-0.8; 2 0,-0.8; 3 0.65,-0.8; 4 0.65,0.8; 5 -0.65,0.8
0402-TIGHT = smd 0.6 x 0.6: 1 -0.5,0; 2 0.5,0
SMA-EDGE = smd 1.5 x 4: GND@0 -2.54,0; GND@1 2.54,0; SIG 0,0 | smd 1.5 x 4 bottom: GND@2 -2.54,0; GND@3 2.54,0
0805 = smd 0.8 x 1.2: 1 -0.9,0; 2 0.9,0
SMT-JUMPER_2_NC_TRACE_SILK = smd 0.66 x 1.27: 1 -0.521,0; 2 0.521,0
STAND-OFF = hole 3.302: 0,0
1X04_NO_SILK = drill 1.016 pad 1.88: 1 0,0; 2 2.54,0; 3 5.08,0; 4 7.62,0
JST-6-SMD-1.25MM-LOCKING = smd 0.6 x 1.7: 1 -3.125,3.3; 2 -1.875,3.3; 3 -0.625,3.3; 4 0.625,3.3; 5 1.875,3.3; 6 3.125,3.3 | smd 1 x 2.7: NC1 4.975,0.1; NC2 -4.975,0.1
MICROSD-EXTERNALPIN = smd 0.7 x 1.6: 1 2.25,10.5; 2 1.15,10.5; 3 0.05,10.5; 4 -1.05,10.5; 5 -2.15,10.5; 6 -3.25,10.5; 7 -4.35,10.5; 8 -5.45,10.5; 9 -6.55,10.5 | smd 1.2 x 1.6: 10 -7.75,9.9 | smd 1.2 x 2.2: 11 -7.75,0.4; 12 7.75,0.4 | smd 1.6 x 1.4: 13 6.85,10 | hole 1: 3.05,0; -4.95,0
1X02_NO_SILK = drill 1.016 pad 1.88: 1 0,0; 2 2.54,0
USB-C-16P_4LAYER-PADS = smd 0.3 x 1: A5 -1.25,-0.34; A6 -0.25,-0.34; A7 0.25,-0.34; A8 1.25,-0.34; B5 1.75,-0.34; B6 0.75,-0.34; B7 -0.75,-0.34; B8 -1.75,-0.34 | smd 0.6 x 1: GND -3.225,-0.34; GND2 3.225,-0.34; VBUS1 -2.45,-0.34; VBUS2 2.45,-0.34 | drill 0.4 pad 0.6 long: SHLD1 -4.318,-0.915; SHLD2 4.318,-0.915; SHLD3 -4.318,-5.095; SHLD4 4.318,-5.095 | hole 0.65: -2.89,-1.445; 2.89,-1.445
1X07_NO_SILK = drill 1.016 pad 1.88: 1 0,0; 2 2.54,0; 3 5.08,0; 4 7.62,0; 5 10.16,0; 6 12.7,0; 7 15.24,0
1X10_NO_SILK = drill 1.016 pad 1.88: 1 0,0; 2 2.54,0; 3 5.08,0; 4 7.62,0; 5 10.16,0; 6 12.7,0; 7 15.24,0; 8 17.78,0; 9 20.32,0; 10 22.86,0
1X06_SOLDER_PADS = smd 3 x 0.9: 1 0,4.445; 2 0,2.667; 3 0,0.889; 4 0,-0.889; 5 0,-2.667; 6 0,-4.445
USB-SOLDER-PADS = smd 3 x 0.9: D+ 0,-0.889; D- 0,0.889; GND 0,-2.667; VBUS 0,2.667
FIDUCIAL-MICRO = smd 0.635 x 0.635: 1 0,0
COMBO-JUMPER_2_NC_TRACE = smd 0.635 x 1.27: 1 -0.508,0; 2 0.508,0 | drill 1.016 pad 1.88: 3 -1.27,0; 4 1.27,0
SOT-416FL = smd 0.46 x 0.65: 1 -0.5,-1.1; 2 0.5,-1.1; 3 0,0.05
TACTILE_SWITCH_SMD_4.6X2.8MM = smd 0.9 x 1: 1 -2.05,-0.8; 2 2.05,-0.8; 3 2.05,0.8; 4 -2.05,0.8
TACTILE_SWITCH_SMD_5.2MM = smd 1.524 x 0.762: 1 -2.794,1.905; 2 2.794,1.905; 3 -2.794,-1.905; 4 2.794,-1.905
RFCMF1220100M4T = smd 0.9 x 0.4: A1 -0.85,0.4; A2 0.85,0.4; B1 -0.85,-0.4; B2 0.85,-0.4
MOSAIC_LGA = smd 0.6 x 0.6: A2 13.97,12.7; A3 13.97,11.43; A4 13.97,10.16; A5 13.97,8.89; A6 13.97,7.62; A7 13.97,6.35; A8 13.97,5.08; A9 13.97,3.81; A10 13.97,2.54; A11 13.97,1.27; A12 13.97,0; A13 13.97,-1.27; A14 13.97,-2.54; A15 13.97,-3.81; A16 13.97,-5.08; A17 13.97,-6.35; A18 13.97,-7.62; A19 13.97,-8.89; A20 13.97,-10.16; A21 13.97,-11.43; A22 13.97,-12.7; A23 13.97,-13.97; AA1 -11.43,13.97; AA2 -11.43,12.7; AA3 -11.43,11.43; AA4 -11.43,10.16; AA5 -11.43,8.89; AA6 -11.43,7.62; AA7 -11.43,6.35; AA8 -11.43,5.08; AA9 -11.43,3.81; AA10 -11.43,2.54; AA11 -11.43,1.27; AA12 -11.43,0; AA13 -11.43,-1.27; AA14 -11.43,-2.54; AA15 -11.43,-3.81; AA16 -11.43,-5.08; AA17 -11.43,-6.35; AA18 -11.43,-7.62; AA19 -11.43,-8.89; AA20 -11.43,-10.16; AA21 -11.43,-11.43; AA22 -11.43,-12.7; AA23 -11.43,-13.97; AB1 -12.7,13.97; AB2 -12.7,12.7; AB3 -12.7,11.43; AB4 -12.7,10.16; AB5 -12.7,8.89; AB6 -12.7,7.62; AB7 -12.7,6.35; AB8 -12.7,5.08; AB9 -12.7,3.81; AB10 -12.7,2.54; AB11 -12.7,1.27; AB12 -12.7,0; AB13 -12.7,-1.27; AB14 -12.7,-2.54; AB15 -12.7,-3.81; AB16 -12.7,-5.08; AB17 -12.7,-6.35; AB18 -12.7,-7.62; AB19 -12.7,-8.89; AB20 -12.7,-10.16; AB21 -12.7,-11.43; AB22 -12.7,-12.7; AB23 -12.7,-13.97; AC1 -13.97,13.97; AC2 -13.97,12.7; AC3 -13.97,11.43; AC4 -13.97,10.16; AC5 -13.97,8.89; AC6 -13.97,7.62; AC7 -13.97,6.35; AC8 -13.97,5.08; AC9 -13.97,3.81; AC10 -13.97,2.54; AC11 -13.97,1.27; AC12 -13.97,0; AC13 -13.97,-1.27; AC14 -13.97,-2.54; AC15 -13.97,-3.81; AC16 -13.97,-5.08; AC17 -13.97,-6.35; AC18 -13.97,-7.62; AC19 -13.97,-8.89; AC20 -13.97,-10.16; AC21 -13.97,-11.43; AC22 -13.97,-12.7; AC23 -13.97,-13.97; B1 12.7,13.97; B2 12.7,12.7; B3 12.7,11.43; B4 12.7,10.16; B5 12.7,8.89; B6 12.7,7.62; B7 12.7,6.35; B8 12.7,5.08; B9 12.7,3.81; B10 12.7,2.54; B11 12.7,1.27; B12 12.7,0; B13 12.7,-1.27; B14 12.7,-2.54; B15 12.7,-3.81; B16 12.7,-5.08; B17 12.7,-6.35; B18 12.7,-7.62; B19 12.7,-8.89; B20 12.7,-10.16; B21 12.7,-11.43; B22 12.7,-12.7; B23 12.7,-13.97; C1 11.43,13.97; C2 11.43,12.7; C3 11.43,11.43; C4 11.43,10.16; C5 11.43,8.89; C6 11.43,7.62; C7 11.43,6.35; C8 11.43,5.08; C9 11.43,3.81; C10 11.43,2.54; C11 11.43,1.27; C12 11.43,0; C13 11.43,-1.27; C14 11.43,-2.54; C15 11.43,-3.81; C16 11.43,-5.08; C17 11.43,-6.35; C18 11.43,-7.62; C19 11.43,-8.89; C20 11.43,-10.16; C21 11.43,-11.43; C22 11.43,-12.7; C23 11.43,-13.97; D1 10.16,13.97; D2 10.16,12.7; D3 10.16,11.43; D21 10.16,-11.43; D22 10.16,-12.7; D23 10.16,-13.97; E1 8.89,13.97; E2 8.89,12.7; E3 8.89,11.43; E21 8.89,-11.43; E22 8.89,-12.7; E23 8.89,-13.97; F1 7.62,13.97; F2 7.62,12.7; F3 7.62,11.43; F21 7.62,-11.43; F22 7.62,-12.7; F23 7.62,-13.97; G1 6.35,13.97; G2 6.35,12.7; G3 6.35,11.43; G21 6.35,-11.43; G22 6.35,-12.7; G23 6.35,-13.97; H1 5.08,13.97; H2 5.08,12.7; H3 5.08,11.43; H21 5.08,-11.43; H22 5.08,-12.7; H23 5.08,-13.97; J1 3.81,13.97; J2 3.81,12.7; J3 3.81,11.43; J21 3.81,-11.43; J22 3.81,-12.7; J23 3.81,-13.97; K1 2.54,13.97; K2 2.54,12.7; K3 2.54,11.43; K21 2.54,-11.43; K22 2.54,-12.7; K23 2.54,-13.97; L1 1.27,13.97; L2 1.27,12.7; L3 1.27,11.43; L21 1.27,-11.43; L22 1.27,-12.7; L23 1.27,-13.97; M1 0,13.97; M2 0,12.7; M3 0,11.43; M21 0,-11.43; M22 0,-12.7; M23 0,-13.97; N1 -1.27,13.97; N2 -1.27,12.7; N3 -1.27,11.43; N21 -1.27,-11.43; N22 -1.27,-12.7; N23 -1.27,-13.97; P1 -2.54,13.97; P2 -2.54,12.7; P3 -2.54,11.43; P21 -2.54,-11.43; P22 -2.54,-12.7; P23 -2.54,-13.97; R1 -3.81,13.97; R2 -3.81,12.7; R3 -3.81,11.43; R21 -3.81,-11.43; R22 -3.81,-12.7; R23 -3.81,-13.97; T1 -5.08,13.97; T2 -5.08,12.7; T3 -5.08,11.43; T21 -5.08,-11.43; T22 -5.08,-12.7; T23 -5.08,-13.97; U1 -6.35,13.97; U2 -6.35,12.7; U3 -6.35,11.43; U21 -6.35,-11.43; U22 -6.35,-12.7; U23 -6.35,-13.97; V1 -7.62,13.97; V2 -7.62,12.7; V3 -7.62,11.43; V21 -7.62,-11.43; V22 -7.62,-12.7; V23 -7.62,-13.97; W1 -8.89,13.97; W2 -8.89,12.7; W3 -8.89,11.43; W21 -8.89,-11.43; W22 -8.89,-12.7; W23 -8.89,-13.97; Y1 -10.16,13.97; Y2 -10.16,12.7; Y3 -10.16,11.43; Y21 -10.16,-11.43; Y22 -10.16,-12.7; Y23 -10.16,-13.97
SOT23-5 = smd 0.55 x 1.2: 1 -0.95,-1.3; 2 0,-1.3; 3 0.95,-1.3; 4 0.95,1.3; 5 -0.95,1.3

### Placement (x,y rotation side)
ANT_V  43.18,31.75 0 bottom
C1  17.78,25.4 0 top
C3  43.18,48.26 90 top
C4  55.24,18.41 0 top
C5  17.78,27.94 0 top
C11  13.97,26.67 0 top
C12  13.97,24.77 180 top
C13  17.78,18.41 180 top
C18  17.78,40.64 0 top
C19  17.78,35.56 0 top
C20  17.78,38.1 0 top
D1  10.16,10.16 90 top
D2  50.8,42.42 0 top
D3  8.89,26.67 180 top
D4  50.8,47.75 0 top
D5  50.8,45.97 0 top
D6  8.89,16.51 180 top
D7  50.8,49.53 0 top
D8  50.8,44.2 0 top
D9  23.37,42.93 90 top
D10  54.61,35.05 270 top
D11  8.89,21.59 270 top
D12  31.75,7.62 270 top
D13  21.59,7.62 270 top
D14  41.91,7.62 270 top
E1  59.69,35.56 270 top
E2  59.69,15.24 270 top
F1  15.24,21.59 90 top
FRAME2  not placed on the board
GP1  43.18,41.91 0 bottom
GP2  43.18,39.37 0 bottom
H1  60.96,48.26 0 top
H2  2.54,48.26 0 top
H3  60.96,2.54 0 top
H4  2.54,2.54 0 top
J1  25.4,1.27 0 top
J2  1.27,21.59 270 top
J3  3.81,35.56 270 top
J4  10.16,1.27 0 top
J5  6.35,10.16 270 top
J6  40.64,1.27 0 top
J7  17.78,49.53 0 top
J8  38.1,1.27 180 top
J9  15.24,1.27 0 top
J12  1.65,21.59 0 bottom
JP1  1.65,10.16 0 bottom
JP21  62.87,50.16 0 top
JP61  0.64,0.64 0 top
JP71  62.87,50.16 0 bottom
JP81  0.64,0.64 0 bottom
LOG  43.18,44.45 0 bottom
LOGO1  SFE_LOGO_NAME_FLAME10_MM  [SFE_LOGO_NAME_FLAME_10MM]  20.32,13.59 0 bottom
LOGO2  6.35,3.81 0 bottom
LOGO4  57.53,6.22 0 top
MEAS  12.7,21.59 270 bottom
PPS  43.18,46.99 0 bottom
PWR  43.18,49.53 0 bottom
Q9  59.69,21.59 90 top
R1  17.78,30.48 180 top
R2  17.78,33.02 0 top
R3  17.78,43.18 0 top
R4  46.99,44.2 180 top
R5  55.24,12.06 0 top
R6  55.24,20.32 0 top
R7  55.24,22.23 0 top
R8  15.24,47.62 270 top
R9  46.99,42.42 180 top
R10  46.99,49.53 180 top
R11  46.99,47.75 180 top
R12  46.99,45.97 180 top
R13  43.18,43.18 270 top
R14  49.53,7.62 0 top
R16  10.16,6.99 180 top
R17  10.16,13.34 180 top
R46  62.23,21.59 270 top
R47  58.42,21.59 270 top
S1  15.24,12.7 270 top
S2  10.16,47.62 180 top
T1  19.05,15.24 0 top
TP1  50.8,7.62 90 bottom
U1  36.83,25.4 180 top
U2  55.24,15.24 270 top
U5  17.78,21.59 0 top
U$1  [V0]  4.19,26.04 0 bottom
U$2  not placed on the board
U$3  [GNSS_1]  31.37,21.59 0 bottom
U$4  [TRIBAND_2]  31.24,25.4 0 bottom
U$5  [MEAS0]  14.61,21.59 270 bottom
U$6  [_ACTIVE_ANT1]  57.28,40.39 0 top
U$7  [#RTK#0]  45.72,3.94 90 top
U$8  [C4]  4.19,20.7 0 bottom
U$9  [D#2]  4.57,10.79 0 bottom
U$10  [D#3]  4.57,9.53 0 bottom
U$11  [G0]  4.95,8.26 0 bottom
U$12  [R5]  4.19,18.92 0 bottom
U$13  [RST0]  17.78,12.7 90 top
U$14  [RX7]  4.7,24.26 0 bottom
U$15  [TX6]  4.83,22.48 0 bottom
U$16  [V8]  4.95,12.06 0 bottom
U$17  [#EVENTA#0]  53.34,5.46 270 bottom
U$18  [COM30]  6.86,21.46 270 bottom
U$19  [MOSAIC#X50]  58.17,29.34 0 top
U$20  [MOSAIC#X5_0]  31.37,29.21 0 bottom
U$21  [TIME0]  55.88,10.79 0 top
U$22  [G1]  4.19,17.14 0 bottom
U$23  [3V30]  46.48,31.75 0 bottom
U$24  [5V0]  40.26,31.75 0 bottom
U$25  [PULSE1]  59.82,10.79 0 top
U$26  [#ANT_V#0]  43.31,33.53 0 bottom
U$27  [#RTK_LED#0]  48.26,39.37 0 bottom
U$28  [RTK0]  54.61,42.42 0 top
U$29  [PVT0]  54.74,44.2 0 top
U$30  [#GP1_#0]  40.64,3.56 270 bottom
U$31  [LOG0]  10.29,44.2 0 top
U$33  [#GP2_#0]  43.18,3.68 270 bottom
U$34  [#PPS_#0]  50.8,3.56 270 bottom
U$35  [#LOG_BTN#0]  48.26,6.1 270 bottom
U$36  [#LOG_L#0]  38.1,45.85 90 top
U$37  [#RDY#0]  33.02,46.74 270 bottom
U$38  [#GP_LED#0]  35.56,45.21 270 bottom
U$39  [#LOG_LED#0]  38.1,44.7 270 bottom
U$40  [#PMIC#0]  40.64,46.48 270 bottom
U$41  [#RTS#0]  20.32,3.81 270 bottom
U$42  [#RTS#0]  30.48,3.81 270 bottom
U$43  [#RTK_#0]  45.72,3.68 270 bottom
U$44  [#EVENTB#0]  55.88,5.46 270 bottom
U$45  [MADE_IN_THE_USA0]  19.05,11.43 0 bottom
U$69  [L1#2#50]  59.05,41.66 0 top
U$79  [LOG2]  54.61,45.97 0 top
U$80  [PPS0]  54.48,47.75 0 top
U$81  [PWR3]  54.74,49.53 0 top
U$82  [COM30]  6.35,21.59 90 top
U$83  [COM20]  27.94,7.62 0 top
U$84  [COM10]  17.78,7.62 0 top
U$85  [COM40]  36.83,7.62 0 top
U$87  [#3#3V#1]  12.7,4.19 90 top
U$88  [#CTS#4]  22.86,3.94 90 top
U$89  [#GND#0]  10.16,4.06 90 top
U$90  [#RTS#5]  20.32,3.94 90 top
U$91  [#RX#2]  15.24,3.56 90 top
U$92  [#TX#3]  17.78,3.56 90 top
U$93  [#3#3V#1]  12.7,4.06 270 bottom
U$94  [#CTS_#4]  22.86,3.68 270 bottom
U$95  [#GND#0]  10.16,3.94 270 bottom
U$97  [#RX_#2]  15.24,3.17 270 bottom
U$98  [#TX_#3]  17.78,3.3 270 bottom
U$99  [COM20]  29.21,7.62 0 bottom
U$100  [#CTS#4]  33.02,3.94 90 top
U$101  [#RTS#5]  30.48,3.94 90 top
U$102  [#RX#2]  25.4,3.56 90 top
U$103  [#TX#3]  27.94,3.56 90 top
U$104  [#CTS_#4]  33.02,3.68 270 bottom
U$106  [#RX_#2]  25.4,3.17 270 bottom
U$107  [#TX_#3]  27.94,3.3 270 bottom
U$108  [COM40]  36.83,7.62 0 bottom
U$109  [COM10]  18.92,7.62 0 bottom
U$110  [#3#3V#1]  20.32,46.74 90 top
U$111  [#RX#2]  35.56,3.56 90 top
U$112  [#TX#3]  38.1,3.56 90 top
U$113  [#GND#0]  17.78,46.86 90 top
U$114  [#3#3V#1]  20.32,46.61 270 bottom
U$115  [#RX_#2]  35.56,3.17 270 bottom
U$116  [#TX_#3]  38.1,3.3 270 bottom
U$117  [#GND#0]  17.78,46.74 270 bottom
U$118  [##RST##2]  30.48,46.99 90 top
U$119  [#GP_LED#4]  35.56,45.34 90 top
U$121  [#PMIC#6]  40.64,46.61 90 top
U$122  [#RDY#3]  33.02,46.86 90 top
U$123  [#VIN#1]  22.86,46.99 90 top
U$124  [#VUSB#0]  25.4,46.35 90 top
U$125  [#V_BAT#7]  27.94,45.59 90 top
U$130  [#VIN#1]  22.86,46.99 270 bottom
U$131  [#VUSB#0]  25.4,46.23 270 bottom
U$132  [#V_BAT#7]  27.94,45.47 270 bottom
U$133  [#_#RST##2]  30.48,46.99 270 bottom
U$134  [L1#2#50]  53.98,35.56 270 bottom
U$135  [_ACTIVE_ANT1]  55.88,35.56 270 bottom
U$136  [TIME0]  53.98,15.24 270 bottom
U$137  [PULSE1]  55.88,15.24 270 bottom
U$138  [GNSS1]  58.17,24.77 0 top
U$140  [TRIBAND2]  58.17,27.05 0 top
U$141  [#LOG_LED#2]  48.26,44.83 0 bottom
U$142  [#PPS_LED#1]  48.13,47.12 0 bottom
U$143  [#GP_LED#3]  47.75,42.42 0 bottom
U$144  [#PWR_LED#0]  48.39,49.53 0 bottom
U$145  [#V_BAT#4]  47.5,36.83 0 bottom
U$146  [#A#8]  53.34,3.05 90 top
U$147  [#B#10]  55.88,2.92 90 top
U$150  [#GP1#0]  40.64,3.81 90 top
U$152  [#GP2#1]  43.18,3.94 90 top
U$154  [#LOG#4]  48.26,4.06 90 top
U$156  [#PPS#6]  50.8,3.81 90 top
VB  43.18,36.83 0 bottom

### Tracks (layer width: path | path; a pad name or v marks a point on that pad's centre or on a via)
1.8V  (via drill 0.3)
  Top/Horz 0.178: U1.AC4 v52.7,13.34 54.83,13.34 R5.2 | R46.2 61.88,21.09 Q9.1 59.83,21.09 v59.56,20.83
  Bottom/Vert 0.178: v59.56,20.83 59.56,24.26 58.29,25.53 53.77,25.53 53.21,24.97 53.21,24.26 54.1,23.37 54.1,14.73 v52.7,13.34
3.3V  (via drill 0.3)
  Top/Horz 0.178: U2.5 56.55,17.2 56.09,17.65 C4.2 56.57,18.41 v57.66,19.51 57.66,19.89 58.42,20.65 R47.2 | U1.C18 v44.21,33.02 | v46.99,23.5 52.83,23.5 v54.1,24.77 | R14.2 v57.15,7.62
  Top/Horz 0.508: C12.2 C11.1 12.06,26.67 11.56,27.18 11.56,29.46 12.57,30.48 R1.2 | U1.B18 U1.C18 U1.C19 U1.C20 | U1.B18 U1.A18 | U1.B18 U1.B19 U1.B20 | U1.A20 U1.A19 U1.A18 | U1.A18 v21.97,33.02 R2.2 | R2.2 18.63,33.95 18.29,34.29 17.14,34.29 16.93,34.51 C19.1 16.93,36.58 | 16.93,36.58 C20.1 C18.1 16.93,41.7 17.14,41.91 18.29,41.91 18.63,42.25 R3.2 18.63,46.7 20.32,48.39 J7.2 | J3.4 16.9,36.61 16.93,36.58 | J4.2 12.7,5.08 v20.32,12.7 | R1.2 16.93,31.41 17.27,31.75 18.16,31.75 18.63,32.22 R2.2 | R1.2 C5.1 C1.1 16.93,24.17 16.83,24.07 U5.5
  Bottom/Vert 0.178: PWR.2 42.66,48.65 43.05,48.26 44.96,48.26 45.72,47.5 45.72,38.09 44.46,36.83 VB.1 43.7,35.31 44.21,34.8 v44.21,33.02 44.2,33.02 44.22,32.99 ANT_V.1 44.22,24.49 45.21,23.5 v46.99,23.5 | v54.1,24.77 56.98,24.77 57.75,24 57.75,19.78 57.66,19.69 v57.66,19.51 56.24,18.09 56.24,8.53 v57.15,7.62
  Bottom/Vert 0.508: v21.97,33.02 22.35,32.64 22.35,14.73 v20.32,12.7
5V  (via drill 0.3)
  Top/Horz 0.305: v42.04,28.57 v42.03,28.58 v20.36,28.58 v20.36,28.57
  Top/Horz 0.508: U5.1 16.83,20.7 | 16.83,20.7 16.83,21.27 17.14,21.59 18.41,21.59 18.73,21.27 U5.3 18.73,19.05 | 18.73,19.05 18.73,18.52 C13.1 | v20.32,19.05 18.73,19.05 | F1.1 15.25,20.7 16.83,20.7
  Bottom/Vert 0.305: v20.32,19.05 20.45,19.18 20.45,28.57 v20.36,28.57 | ANT_V.3 42.14,28.68 v42.04,28.57
!RESET!  (via drill 0.3)
  Top/Horz 0.178: v14.48,13.72 14.99,13.72 16.02,14.75 S1.4 16.04,16.66 16.55,17.16 19.91,17.16 20.95,18.21 20.95,23.5 v21.59,24.13 U1.A11 | v21.59,44.96 23.11,46.48 29.97,46.48 30.48,46.99 J7.6 | D9.3 23.43,43.58 22.93,43.07 21.47,43.07 20.74,42.34 v20.74,42.29 | v14.48,11.65 15.62,11.65 16.04,11.23 S1.3
  Bottom/Vert 0.178: v14.48,13.72 v14.48,11.65 | v21.59,24.13 20.95,24.77 20.95,42.29 | 20.95,42.29 20.95,44.32 v21.59,44.96 | v20.74,42.29 20.95,42.29
ANT_V  (via drill 0.3)
  Top/Horz 0.305: v42.55,35.57 42.55,36.57 42.54,36.57 42.54,39.92 44.24,41.62 44.24,42.97 R13.1 C3.1
  Bottom/Vert 0.305: v42.55,35.57 43.18,34.94 ANT_V.2
CC1
  Top/Horz 0.178: J5.A5 6.71,11.41 8.64,13.34 R17.2
CC2
  Top/Horz 0.178: J5.B5 7.21,8.41 8.64,6.99 R16.2
COM1_CTS
  Top/Horz 0.178: U1.E1 27.94,10.66 24.25,6.97 22.86,6.97 | 22.86,6.97 J9.4 | D13.4 22.86,6.97
COM1_RTS  (via drill 0.3)
  Top/Horz 0.178: U1.C1 23.75,9.78 22.23,9.78 21.42,8.97 21.42,7.12 21.27,6.97 D13.3 20.79,6.57 20.45,6.22 v20.32,6.22
  Bottom/Vert 0.178: v20.32,6.22 J9.3
COM1_RX
  Top/Horz 0.178: U1.B1 22.86,10.16 20.83,10.16 | 20.83,10.16 19.05,10.16 15.24,6.35 J9.1 | D13.1 20.79,10.12 20.83,10.16
COM1_TX
  Top/Horz 0.178: U1.D1 26.67,10.41 24.53,8.27 D13.5 22.01,8.27 21.77,8.03 21.77,6.36 20.5,5.08 19.05,5.08 17.78,3.81 J9.2
COM2_CTS
  Top/Horz 0.178: U1.J1 32.55,10.96 D12.5 33.13,8.27 33.53,7.87 33.53,6.1 33.02,5.59 J1.4
COM2_RTS
  Top/Horz 0.178: J1.3 30.48,5.08 29.46,6.1 29.46,8.26 | U1.G1 30.48,10.41 29.46,9.4 29.46,8.26 | D12.1 29.48,8.27 29.46,8.26
COM2_RX  (via drill 0.3)
  Top/Horz 0.178: U1.F1 29.21,10.79 25.4,6.99 J1.1 | D12.3 31.51,6.97 31.75,6.73 v31.75,5.97
  Bottom/Vert 0.178: v31.75,5.97 31.37,5.59 25.91,5.59 25.4,5.08 J1.1
COM2_TX  (via drill 0.3)
  Top/Horz 0.178: U1.H1 31.75,7.23 32.01,6.97 D12.4 32.55,5.88 v31.75,5.08
  Bottom/Vert 0.178: v31.75,5.08 29.21,5.08 27.94,3.81 J1.2
COM3_CTS  (via drill 0.3)
  Top/Horz 0.178: U1.N1 v38.1,8.26 | D11.4 9.69,20.23 9.4,19.94 6.73,19.94 5.71,20.96 J2.4 2.73,20.96 v1.65,19.88
  Bottom/Vert 0.178: v38.1,8.26 13.89,8.26 6.4,15.74 6.06,15.74 5.08,16.73 5.08,17.82 3.02,19.88 v1.65,19.88 J12.4
COM3_RTS  (via drill 0.3)
  Top/Horz 0.178: U1.L1 v35.56,9.53 | D11.5 10.4,22.24 10.67,21.97 10.67,20.45 9.72,19.49 9.65,19.43 6.35,19.43 | v5.8,17.36 6.35,17.91 6.35,19.43 | v1.65,18.1 3.26,19.71 J2.5 6.07,19.71 6.35,19.43
  Bottom/Vert 0.178: v35.56,9.53 13.63,9.53 6.91,16.25 6.91,16.59 6.56,16.94 6.21,16.94 v5.8,17.36 | v1.65,18.1 J12.5
COM3_RX  (via drill 0.3)
  Top/Horz 0.178: U1.K1 v34.29,10.16 | v1.65,23.44 4.54,23.44 J2.2 5.87,23.46 7.1,22.24 D11.1
  Bottom/Vert 0.178: J12.2 v1.65,23.44 3.02,23.44 4.95,21.5 4.95,19.05 7.26,16.74 7.26,16.39 13.5,10.16 v34.29,10.16
COM3_TX  (via drill 0.3)
  Top/Horz 0.178: U1.M1 v36.83,8.89 | D11.3 7,20.94 5.71,22.23 4.58,22.23 J2.3 4.05,22.21 3.5,21.66 v1.65,21.66 0.76,20.77 0.76,17.78 1.16,17.38 2.94,17.38 3.81,16.51 3.81,15.88 4.11,15.58 5.55,15.58 v6.31,16.34
  Bottom/Vert 0.178: J12.3 v1.65,21.66 | v6.31,16.34 13.76,8.89 v36.83,8.89
COM4_RX  (via drill 0.3)
  Top/Horz 0.178: U1.D3 33.02,20.32 v38.99,20.32 | D14.1 39.21,8.27 35.56,4.62 J8.2
  Bottom/Vert 0.178: J8.2 35.56,3.09 38.86,6.39 38.86,20.19 v38.99,20.32
COM4_TX  (via drill 0.3)
  Top/Horz 0.178: U1.E3 32.89,18.92 v39.62,18.92 | D14.3 38.97,6.97 38.1,6.1 J8.1
  Bottom/Vert 0.178: v39.62,18.92 39.37,18.67 39.37,5.08 38.1,3.81 J8.1
D+
  Top/Horz 0.178: T1.B2 21.19,14.84 U1.A5
D-
  Top/Horz 0.178: T1.A2 20.72,15.64 U1.A6
EVENTA  (via drill 0.3)
  Top/Horz 0.178: R6.2 56.09,20.37 v55.24,21.22
  Bottom/Vert 0.178: J6.6 53.34,9.14 54.52,10.32 54.52,20.61 55.13,21.22 v55.24,21.22
EVENTB  (via drill 0.3)
  Top/Horz 0.178: v56.13,23.37 56.13,22.26 R7.2
  Bottom/Vert 0.178: v56.13,23.37 55.88,23.11 J6.7
GND  (via drill 0.3)
  other vias: 5.08,45.72 19.68,34.8 19.68,31.24 16,26.67 19.56,26.67 13.97,19.05 15.62,19.05 11.94,17.02 4.7,16.26 12.19,13.97 14.48,15.75 13.08,11.56 6.99,14.1 7.11,6.86 12.7,6.99 59.69,19.05 58.42,19.05 57.15,17.78 59.69,11.43 58.42,11.43 60.96,11.43 60.96,13.97 59.69,13.97 58.42,13.97 58.42,16.51 59.69,16.51 60.96,16.51 60.96,19.05 60.96,31.75 59.69,31.75 58.42,31.75 57.15,33.02 58.42,34.16 59.69,34.16 60.96,34.16 60.96,36.96 59.69,36.96 58.42,36.96 57.15,38.1 58.42,39.37 59.69,39.37 60.96,39.37 57.15,31.75 52.96,48.51 52.96,46.74 52.96,44.45 2.54,27.94 40.01,13.34 40.01,15.24 41.4,15.24 40.01,10.29 40.01,12.06 49.53,10.16 47.62,10.16 50.16,15.88 50.16,17.14 48.9,17.14 48.9,15.88 50.16,14.61 50.16,13.34 48.9,20.95 48.9,19.68 48.9,18.41 46.99,35.56 46.99,34.29 46.99,33.02 46.99,31.75 46.99,30.48 46.99,29.21 46.99,27.94 46.99,26.67 52.07,26.67 52.07,27.94 52.07,29.21 52.07,33.02 52.07,31.75 52.07,30.48 52.07,34.29 52.07,36.83 52.07,38.1 52.07,39.37 50.8,40.64 49.53,40.64 46.99,40.64 45.72,35.56 37.47,37.47 37.47,38.61 34.29,40.64 35.56,40.64 32.51,40.64 31.75,35.56 30.48,35.56 29.21,35.56 26.04,37.47 29.84,38.73 31.11,38.73 28.57,38.73 27.3,38.73 27.3,37.47 28.57,37.47 29.84,37.47 31.11,37.47 33.02,35.56 34.29,35.56 35.56,35.56 24.77,36.2 23.5,36.2 23.5,37.47 23.5,38.73 22.1,38.73 22.1,37.47 22.1,36.2 26.04,38.73 26.04,40.01 27.3,40.01 28.57,40.01 29.84,40.01 31.11,40.01 53.21,18.41 52.83,16.38 55.12,14.35 24.77,17.14 23.5,17.14 23.5,18.41 24.77,18.41 23.5,15.88 24.77,15.88 23.5,14.61 27.3,13.34 28.57,13.34 31.11,13.34 34.92,13.34 18.67,39.12 15.75,38.23 23.5,31.11 23.5,29.84 24.77,29.84 24.77,32.26 23.5,32.26 23.5,26.04 19.3,41.78 12.7,8.38 40.01,37.47 41.27,37.47 46.35,37.47 46.35,38.73 47.62,38.73 47.62,37.47 48.9,37.47 50.16,37.47 48.9,36.2 48.9,34.92 48.9,33.66 50.16,33.66 48.9,32.38 48.9,31.11 48.9,29.84 48.9,28.57 48.9,27.3 48.9,38.73 50.16,38.73 41.27,38.73 45.09,38.73 9.02,21.59 25.27,42.93 19.05,6.35 30.48,6.22 42.04,7.62
  pour Top/Horz (isolate 0.203, rank 4): 0,50.8 0,0 63.5,0 63.5,50.8
  pour Bottom/Vert (isolate 0.203, rank 4): 63.5,50.8 63.5,0 0,0 0,50.8
  pour Vert (isolate 0.203, rank 4): 63.5,50.8 63.5,0 0,0 0,50.8
  pour GND/Horz (isolate 0.203, rank 4): 63.5,50.8 63.5,0 0,0 0,50.8
GP1  (via drill 0.3)
  Top/Horz 0.178: v46.99,21.59 46.99,21.42 47.59,20.82 47.59,15.91 U1.AA4 | J6.1 40.64,3.94 42.71,6.01 D14.4
  Bottom/Vert 0.178: v46.99,21.59 41.4,21.59 40.64,20.83 J6.1
GP2  (via drill 0.3)
  Top/Horz 0.178: U1.L3 35.56,15.49 37.08,17.02 v43.18,17.02 | D14.5 43.29,8.27 43.43,8.13 43.43,5.59 43.18,5.33 J6.2
  Bottom/Vert 0.178: J6.2 v43.18,17.02
GPS_ANT1
  Top/Horz 0.349: U1.AC20 D10.1 | D10.1 | D10.1 E1.SIG
LOG_BTN  (via drill 0.3)
  Top/Horz 0.178: U1.K3 34.29,15.24 36.83,17.78 v44.45,17.78 | R8.2 v15.24,44.45 | v46.99,19.05 46.28,19.76 46.28,33.72 45.15,34.85 37.54,34.85 36.2,36.2 36.2,41 35.23,41.96 28.39,41.96 25.8,44.55 22.33,44.55 21.76,43.98 v19.98,43.98 | R14.1 48.68,6.35 48.26,5.93 J6.4
  Bottom/Vert 0.178: 46.99,17.78 46.99,3.81 48.26,2.54 J6.4 | 46.99,17.78 v46.99,19.05 | v44.45,17.78 46.99,17.78 | v15.24,44.45 19.51,44.45 v19.98,43.98
LOG_LED  (via drill 0.3)
  Top/Horz 0.178: U1.B2 24.77,13.34 25.78,13.34 26.04,13.59 26.04,14.22 33.4,21.59 v37.72,21.59 | v39.5,43.18 v39.5,40.64
  Bottom/Vert 0.178: J7.9 38.1,45.72 39.37,44.45 39.5,44.45 | v37.72,21.59 37.72,33.14 39.01,34.44 39.01,38.25 39.5,38.73 v39.5,40.64 | 39.5,44.45 LOG.2 | v39.5,43.18 39.5,44.45
MEAS  (via drill 0.3)
  Top/Horz 0.508: MEAS.4 10.04,17.66 D6.C | D3.C 10.04,24.25 v10.16,24.13
  Bottom/Vert 0.508: MEAS.2 MEAS.4 11.68,20.32 10.16,21.84 v10.16,24.13
MODULE_RDY  (via drill 0.3)
  Top/Horz 0.178: J7.7 33.02,46.99 32,45.97 24.51,45.97 v24.13,45.59 | v21.55,25.4 U1.A12
  Bottom/Vert 0.178: v24.13,45.59 23.62,45.59 21.34,43.31 21.34,25.62 v21.55,25.4
N$1
  Top/Horz 0.178: S2.4 S2.3 14.19,49.53 R8.1
N$2
  Top/Horz 0.178: D4.A R11.1
N$3  (via drill 0.3)
  Top/Horz 0.178: R11.2 44.7,47.75 v44.58,47.62
  Bottom/Vert 0.178: v44.58,47.62 43.95,47.62 43.7,47.37 PPS.1
N$4
  Top/Horz 0.508: MEAS.3 13.59,22.86 13.97,22.48 15.23,22.48 F1.2
  Bottom/Vert 0.508: MEAS.1 MEAS.3
N$5  (via drill 0.3)
  Top/Horz 0.178: R1.1 19.56,29.55 v19.56,29.21 | v12.7,34.29 12.82,34.41 J3.2
  Bottom/Vert 0.178: v19.56,29.21 17.78,29.21 v12.7,34.29
N$6
  Top/Horz 0.178: U1.AC6 53.34,20.32 R6.1
N$7
  Top/Horz 0.178: U1.AC7 51.18,19.05 54.36,22.23 R7.1
N$8
  Top/Horz 0.178: R9.1 D2.A
N$9  (via drill 0.3)
  Top/Horz 0.178: v45.09,41.02 45.09,41.36 R9.2
  Bottom/Vert 0.178: GP2.1 43.7,39.64 v45.09,41.02
N$10
  Top/Horz 0.305: U1.AC17 U1.AC16
N$11
  Top/Horz 0.178: D8.A R4.1
N$12  (via drill 0.3)
  Top/Horz 0.178: v45.09,43.56 45.51,43.56 R4.2
  Bottom/Vert 0.178: v45.09,43.56 43.7,42.18 GP1.1
N$14
  Top/Horz 0.178: R10.1 D7.A
N$15
  Top/Horz 0.305: U1.M23 U1.N23
N$16
  Top/Horz 0.178: D5.A R12.1
N$17  (via drill 0.3)
  Top/Horz 0.178: R12.2 44.7,45.97 v44.45,45.72
  Bottom/Vert 0.178: v44.45,45.72 44.45,45.47 43.7,44.72 LOG.1
N$20  (via drill 0.3)
  Top/Horz 0.178: R10.2 v44.58,49.53
  Bottom/Vert 0.178: v44.58,49.53 PWR.1
N$26
  Top/Horz 0.178: U1.AC3 52.7,12.06 R5.1
PMIC_ON_REQ  (via drill 0.3)
  Top/Horz 0.178: J7.10 40.64,46.99 38.73,45.09 v26.67,45.09 | v26.71,31.11 24.77,31.11 U1.B16
  Bottom/Vert 0.178: v26.67,45.09 26.67,31.11 v26.71,31.11
PPS  (via drill 0.3)
  Top/Horz 0.178: E2.SIG 57.4,15.24 57.15,14.99 57.15,14.35 | 57.15,14.35 57.15,11.05 56.26,10.16 v50.8,10.16 | U2.4 56.61,14.35 57.15,14.35
  Bottom/Vert 0.178: TP1.2 v50.8,10.16
PPS_1V8
  Top/Horz 0.178: U1.AC8 54.61,24.13 61.59,24.13 62.23,23.5 R46.1 61.88,22.09 Q9.2
PPS_3
  Top/Horz 0.178: Q9.3 59.27,21.59 R47.1 57.49,22.44 57.15,22.1 57.15,19.89 56.69,19.43 53.09,19.43 52.07,18.41 52.07,15.88 52.7,15.24 U2.2
PPS_3V3  (via drill 0.3)
  Top/Horz 0.178: v41.78,46.99 41.78,47.75 42.32,48.29 43.79,48.29 44.14,48.64 48.77,48.64 v48.9,48.51
  Bottom/Vert 0.178: PPS.2 v41.78,46.99 | v48.9,48.51 48.9,46.35 48.26,45.72 48.26,7.37 48.53,7.1 TP1.1 J6.5
PVT_LED  (via drill 0.3)
  Top/Horz 0.178: v36.83,27.3 23.5,27.3 U1.A14
  Bottom/Vert 0.178: v36.83,27.3 36.2,27.94 36.2,41.91 | 36.2,41.91 36.2,42.55 35.56,43.18 J7.8 | GP1.2 36.2,41.91
RTK_LED  (via drill 0.3)
  Top/Horz 0.178: v45.72,15.24 45.72,15.32 44.82,16.22 39.08,16.22 v38.1,15.24 U1.M3
  Bottom/Vert 0.178: GP2.2 40.64,39.37 39.37,38.1 39.37,34.29 38.14,33.06 38.14,22.4 38.32,22.22 38.32,15.46 v38.1,15.24 | J6.3 v45.72,15.24
SD_CLK  (via drill 0.3)
  Top/Horz 0.178: J3.5 v12.7,37.72 | U1.AA1 47.68,12.01 47.68,14.33 46.71,15.3 46.71,16.91 45.57,18.05 45.57,33.42 44.85,34.14 34.7,34.14 33.66,35.18 33.66,40.36 32.77,41.25 26.31,41.25 v26.07,41.49 | v17.78,39.46 18.16,39.84 19.14,39.84 19.31,39.66 20.41,39.66 22.06,41.31 v22.06,41.44 22.12,41.38 22.57,41.82 D9.5
  Bottom/Vert 0.178: v17.78,39.46 17.27,39.46 16.15,40.58 13.15,40.58 12.7,40.13 v12.7,37.72 | v26.07,41.49 22.11,41.49 v22.06,41.44
SD_CMD  (via drill 0.3)
  Top/Horz 0.178: R2.1 16.26,33.02 15.75,33.53 v15.75,34.54 15.75,35.05 15.29,35.51 J3.3 | U1.AB1 48.95,12.01 48.95,14.08 48.37,14.66 47.95,14.66 47.07,15.54 47.07,17.06 45.92,18.2 45.92,33.57 45,34.49 35.74,34.49 34.92,35.31 34.92,40.89 34.21,41.6 28.25,41.6 25.65,44.2 22.86,44.2 22.57,43.9 D9.4 20.59,43.58 20.07,43.05 20.07,40.76 v19.69,40.39
  Bottom/Vert 0.178: v15.75,34.54 17.44,36.23 18.79,36.23 19.94,37.39 19.94,40.13 v19.69,40.39
SD_DATA  (via drill 0.3)
  Top/Horz 0.178: J3.7 15.72,39.91 | 15.72,39.91 v15.75,39.88 | R3.1 15.72,41.97 15.72,39.91 | U1.Y1 46.35,12.06 46.35,16.76 45.21,17.91 45.21,33.27 44.7,33.78 33.53,33.78 32.38,34.92 32.38,39.62 31.11,40.89 25.02,40.89 | v17.78,36.83 19.3,36.83 20.45,37.97 20.45,38.73 22.61,40.89 25.02,40.89 | D9.1 24.78,42.28 25.02,42.04 25.02,40.89
  Bottom/Vert 0.178: v15.75,39.88 15.75,39.37 17.78,37.34 v17.78,36.83
USB_D+  (via drill 0.3)
  Top/Horz 0.178: J5.A6 5.2,10.41 4.95,10.16 4.95,9.53 5.08,9.4 6,9.4 J5.B6 7.23,9.41 v7.43,9.21 D1.6 9.85,9.21 10.16,9.53 10.16,11.18 11.2,12.21 13.1,12.21 13.54,12.66 16.21,12.66 16.32,12.76 17.4,13.84 17.4,14.61 17.65,14.86 18.18,14.86 T1.B1
  Bottom/Vert 0.178: JP1.D+ 7.37,9.27 v7.43,9.21
USB_D-  (via drill 0.3)
  Top/Horz 0.178: J5.B7 6.86,10.91 | 6.86,10.91 6.99,10.91 7.11,11.04 v7.48,11.04 7.55,11.11 D1.4 9.59,11.11 11.05,12.57 12.95,12.57 13.4,13.02 16.07,13.02 17.04,13.99 17.04,15.27 17.42,15.64 T1.A1 | J5.A7 6.74,9.91 6.86,10.03 6.86,10.91
  Bottom/Vert 0.178: JP1.D- v7.47,11.05 v7.48,11.04
V_BAT  (via drill 0.3)
  Top/Horz 0.178: v27.94,19.81 27.88,19.75 24.66,19.75 24.13,20.28 U1.B8 | v38.73,31.75 v27.94,31.75
  Bottom/Vert 0.178: J7.5 v27.94,31.75 v27.94,19.81 | VB.2 41.01,36.83 40.12,35.94 40.12,34.53 38.73,33.15 v38.73,31.75
V_USB  (via drill 0.3)
  Top/Horz 0.305: J5.VBUS2 5.39,7.71 4.32,8.78 4.32,11.54 5.39,12.61 J5.VBUS1 | U1.A8 v21.59,20.32
  Top/Horz 0.508: 7.43,12.89 7.15,12.61 J5.VBUS1 | 7.43,12.89 7.75,13.2 D6.A 7.74,17.66 v7.62,17.78 | v7.39,12.93 7.43,12.89 | D1.5 v7.49,10.16
  Bottom/Vert 0.305: v21.59,20.32 21.59,19.05 20.32,17.78 v7.62,17.78
  Bottom/Vert 0.508: J7.4 25.4,48.26 22.86,45.72 10.16,45.72 8.89,44.45 8.89,26.67 7.24,25.02 7.24,18.16 v7.62,17.78 | JP1.VBUS 3.42,12.83 4.21,12.04 6.5,12.04 v7.39,12.93 8.24,12.08 8.24,10.47 7.94,10.16 v7.49,10.16
VANT
  Top/Horz 0.305: U1.P23 U1.R23 40.64,40.64 42.33,42.33 R13.2
VIN  (via drill 0.3)
  Top/Horz 0.508: J2.1 7.19,24.71 7.75,25.27 D3.A 7.74,27.82 v7.62,27.94
  Bottom/Vert 0.508: J7.3 22.86,48.26 21.59,46.99 10.16,46.99 7.44,44.27 7.44,28.12 v7.62,27.94 5.71,26.04 J12.1

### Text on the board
GND/Horz: 2
Vert: 15
Bottom/Vert: v11
Measures: All dimensions in inches.
tDocu: Solder Mask: Red | Layers: 4 | Controlled Impedance: JLC7628 | Finish: ENIG | Thickness: 1.6mm | No clean process | Material: TG155 | N. Seidle

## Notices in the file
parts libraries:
SparkFun-Resistors: Licensing: Creative Commons ShareAlike 4.0 International - https://creativecommons.org/licenses/by-sa/4.0
SparkFun-Aesthetics: Released under the Creative Commons Attribution Share-Alike 4.0 License
SparkFun-Aesthetics: https://creativecommons.org/licenses/by-sa/4.0
